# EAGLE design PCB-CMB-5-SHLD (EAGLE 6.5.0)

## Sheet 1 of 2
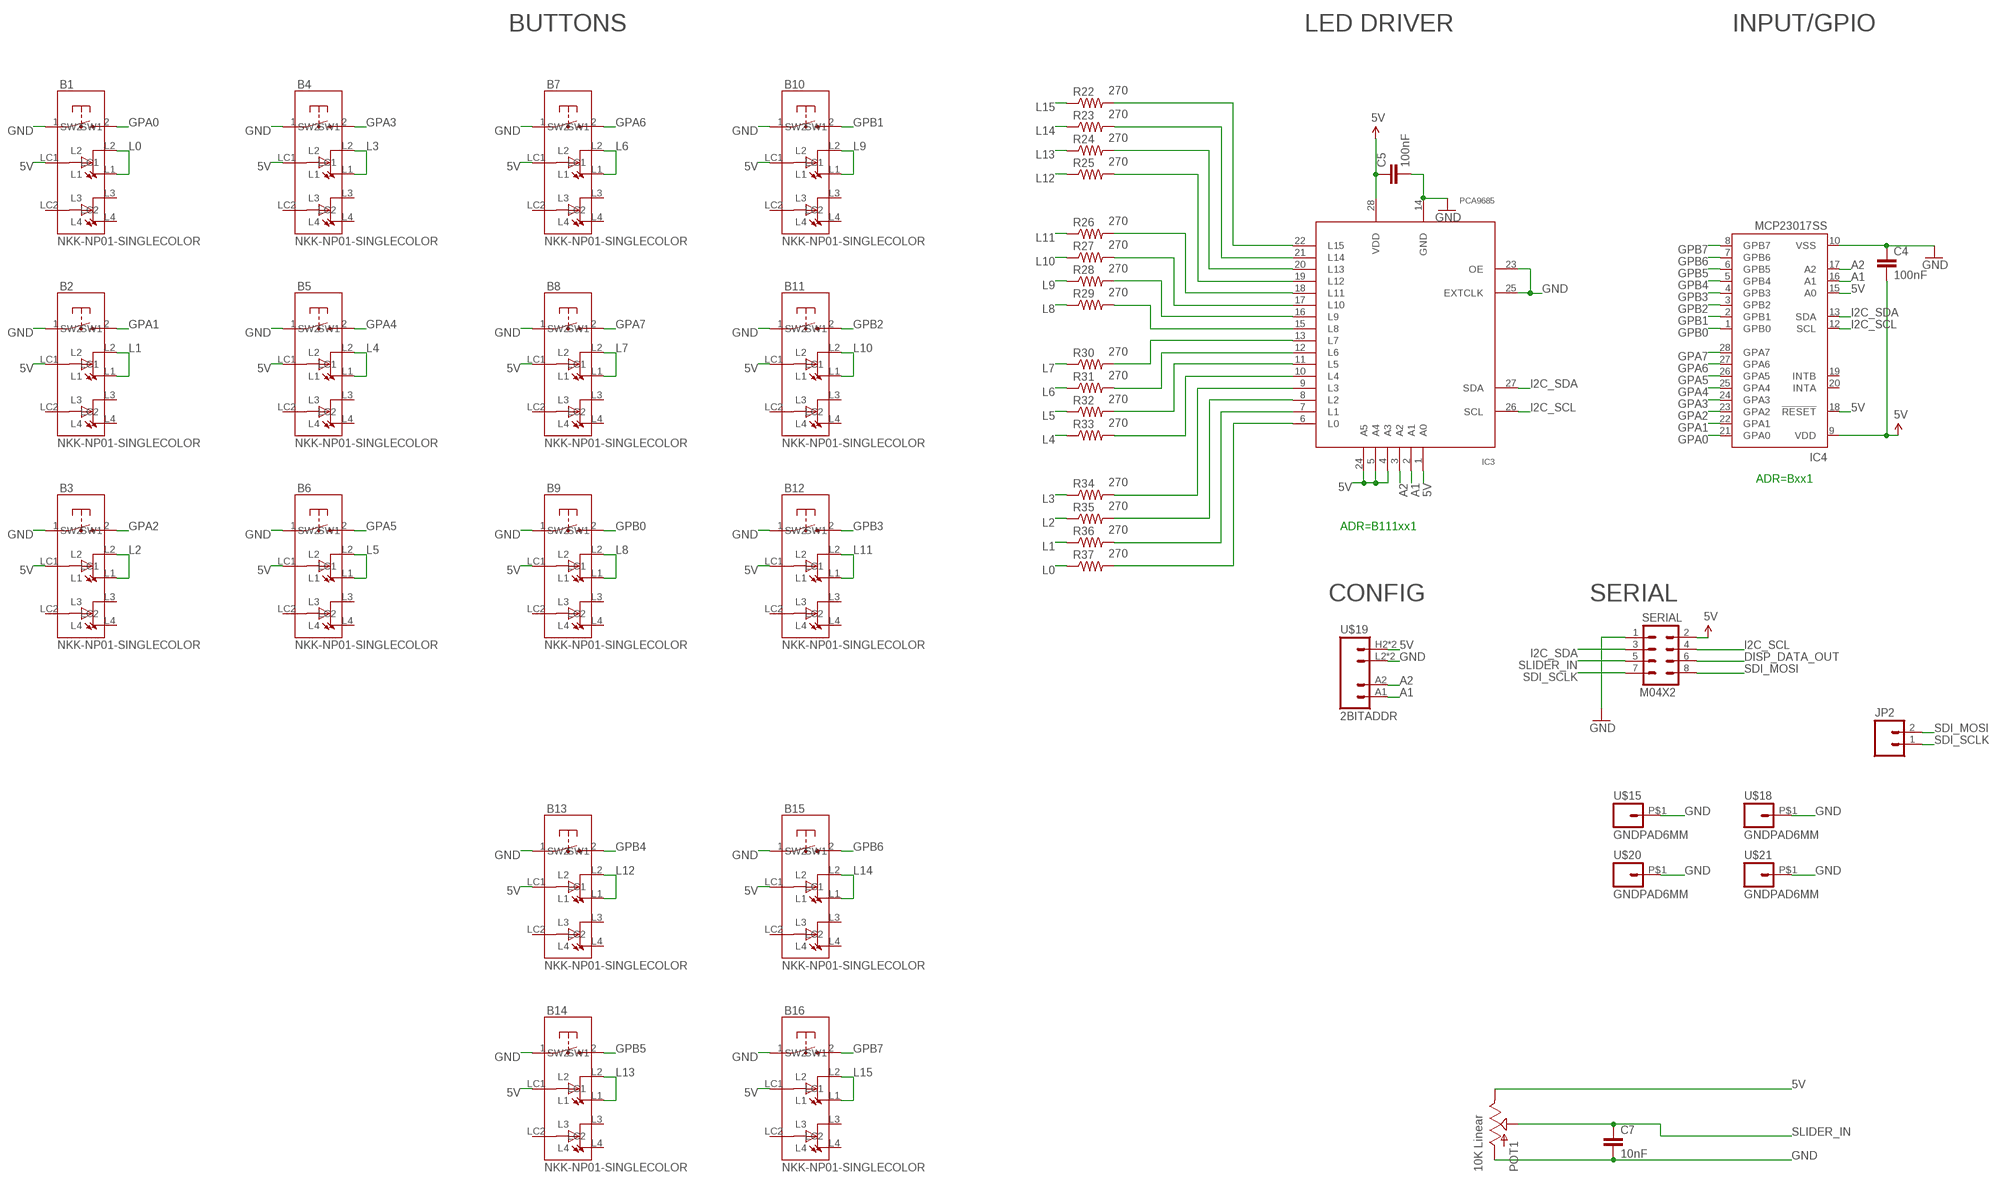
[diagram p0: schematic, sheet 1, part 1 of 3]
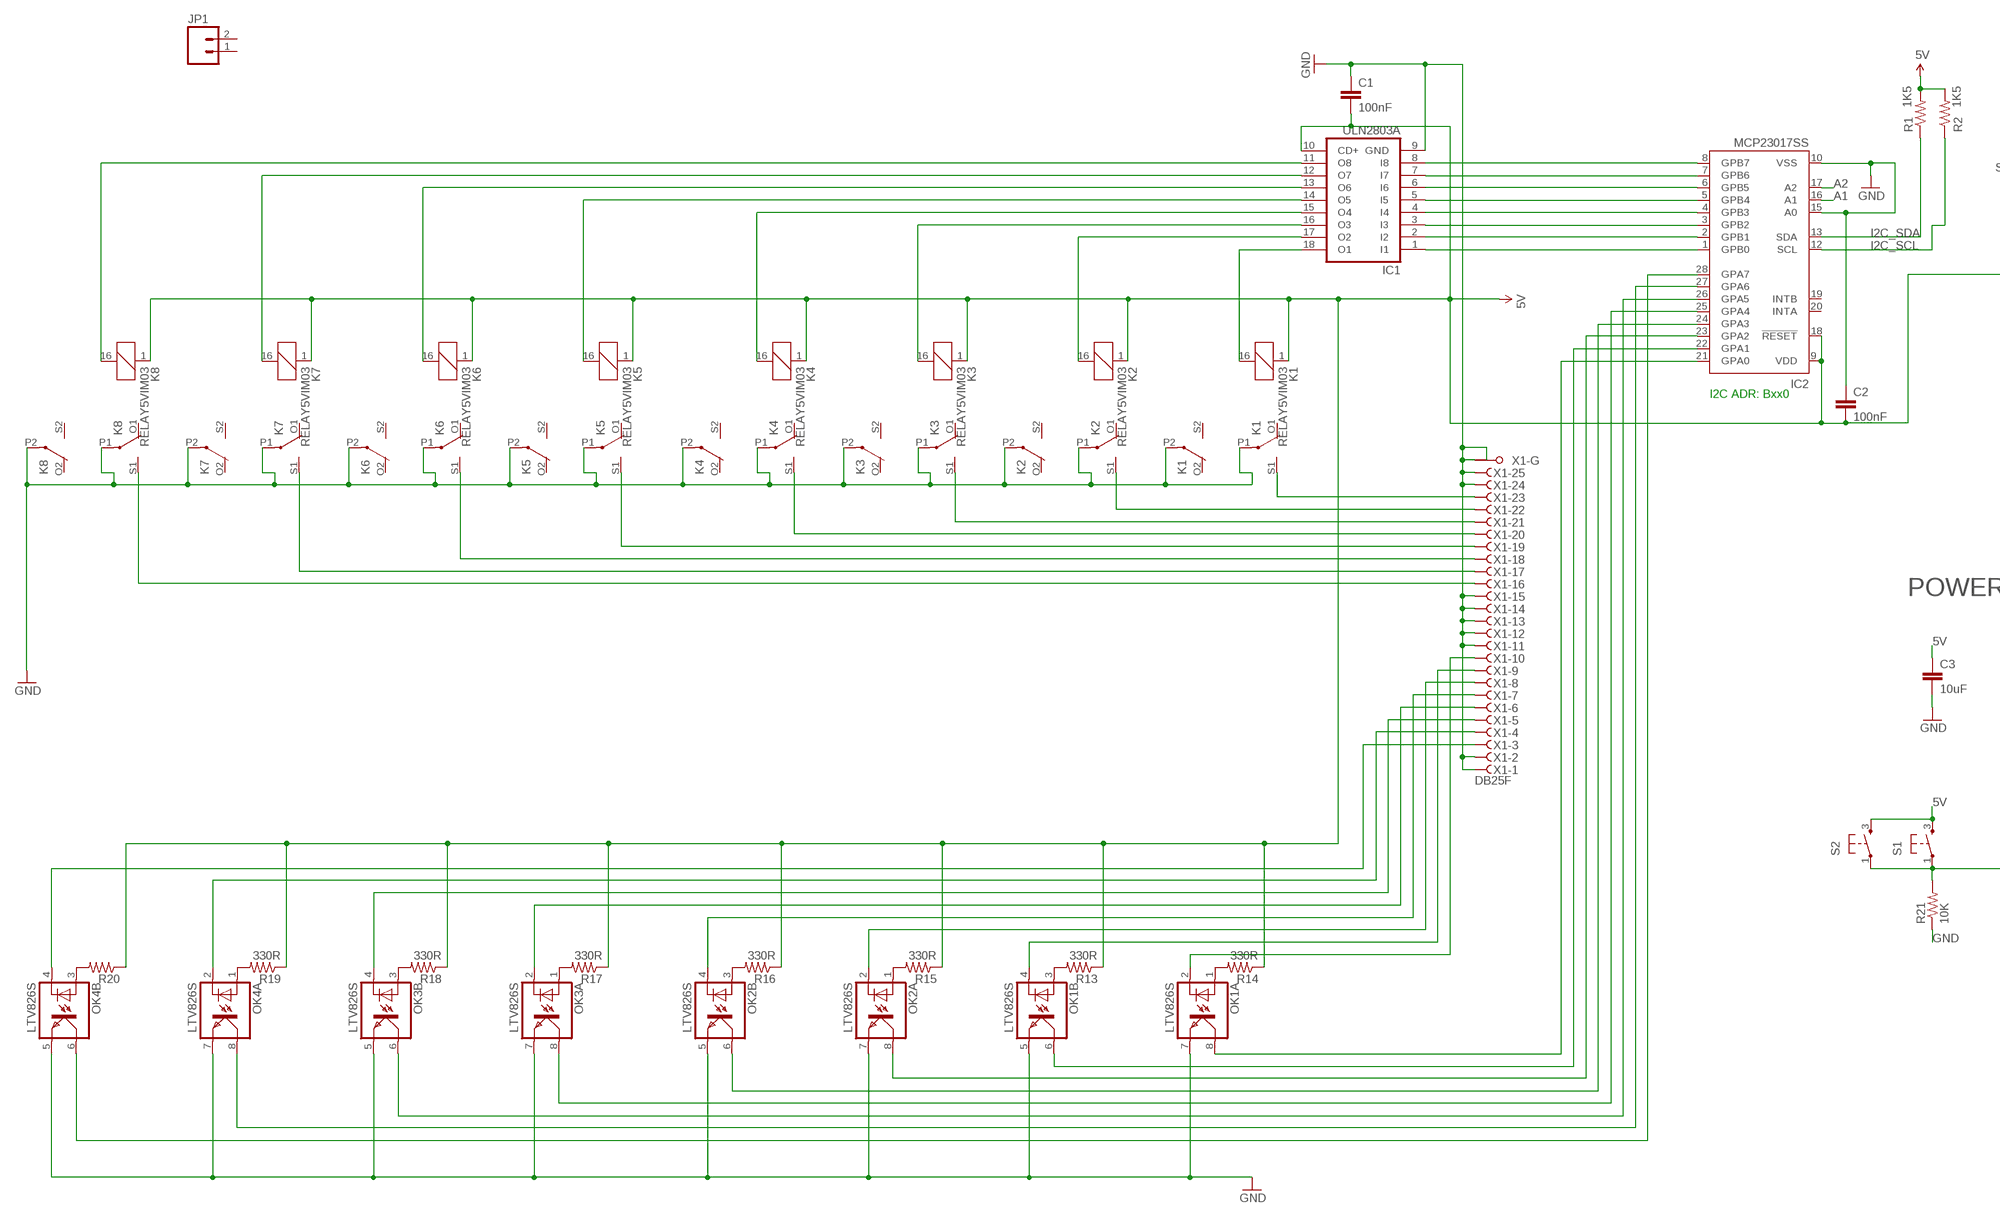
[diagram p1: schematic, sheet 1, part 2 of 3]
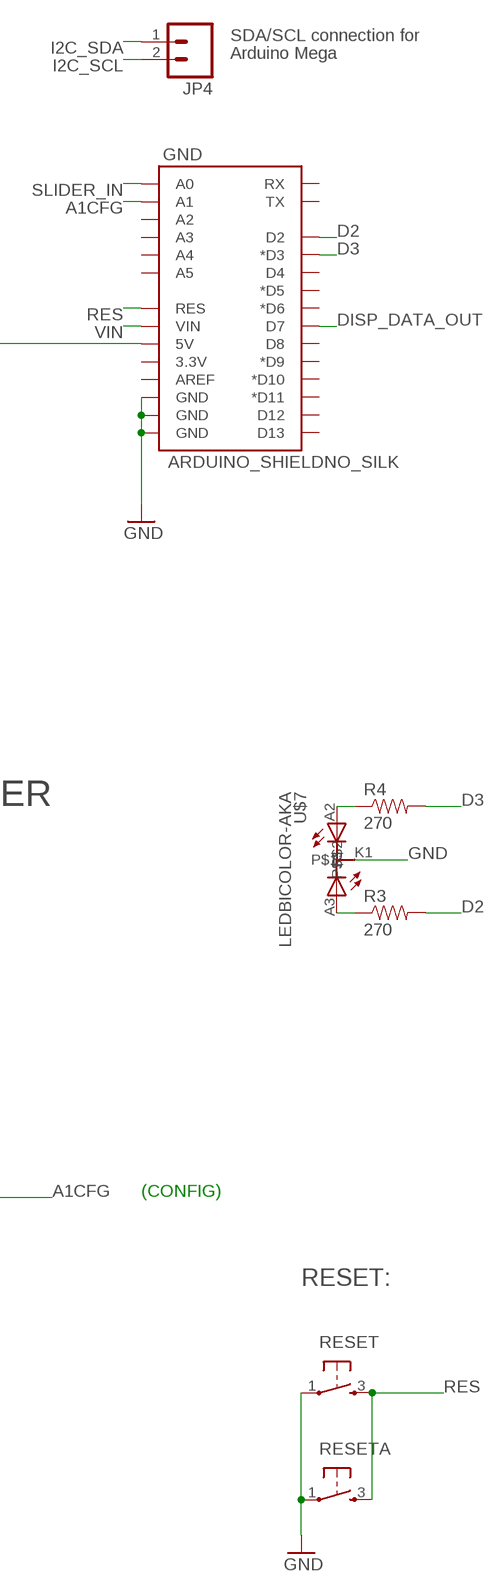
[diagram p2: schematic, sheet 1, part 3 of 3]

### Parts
B1  NKK-NP01-SINGLECOLOR  [NKK-NP01]
B2  NKK-NP01-SINGLECOLOR  [NKK-NP01]
B3  NKK-NP01-SINGLECOLOR  [NKK-NP01]
B4  NKK-NP01-SINGLECOLOR  [NKK-NP01]
B5  NKK-NP01-SINGLECOLOR  [NKK-NP01]
B6  NKK-NP01-SINGLECOLOR  [NKK-NP01]
B7  NKK-NP01-SINGLECOLOR  [NKK-NP01]
B8  NKK-NP01-SINGLECOLOR  [NKK-NP01]
B9  NKK-NP01-SINGLECOLOR  [NKK-NP01]
B10  NKK-NP01-SINGLECOLOR  [NKK-NP01]
B11  NKK-NP01-SINGLECOLOR  [NKK-NP01]
B12  NKK-NP01-SINGLECOLOR  [NKK-NP01]
B13  NKK-NP01-SINGLECOLOR  [NKK-NP01]
B14  NKK-NP01-SINGLECOLOR  [NKK-NP01]
B15  NKK-NP01-SINGLECOLOR  [NKK-NP01]
B16  NKK-NP01-SINGLECOLOR  [NKK-NP01]
C1  100nF  CAP0805  [0805]
C2  100nF  CAP0603-CAP  [0603-CAP]
C3  10uF  CAP0805  [0805]
C4  100nF  CAP0603-CAP  [0603-CAP]
C5  100nF  CAP0603-CAP  [0603-CAP]
C7  10nF  CAP0603-CAP  [0603-CAP]
GND  ARDUINO_SHIELDNO_SILK  [DUEMILANOVE_VIAS]
IC1  ULN2803A  ULN2803ASO18W  [SO18W]
IC2  MCP23017SS  [SSOP28]
IC3  PCA9685  [TSSOP28]
IC4  MCP23017SS  [SSOP28]
JP1  M02PTH  [1X02]
JP2  M02PTH  [1X02]
JP4  M02PTH  [1X02]
K1  RELAY5VIM03  [DS2Y]
K2  RELAY5VIM03  [DS2Y]
K3  RELAY5VIM03  [DS2Y]
K4  RELAY5VIM03  [DS2Y]
K5  RELAY5VIM03  [DS2Y]
K6  RELAY5VIM03  [DS2Y]
K7  RELAY5VIM03  [DS2Y]
K8  RELAY5VIM03  [DS2Y]
OK1  LTV826S  [DIL8-SMD]
OK2  LTV826S  [DIL8-SMD]
OK3  LTV826S  [DIL8-SMD]
OK4  LTV826S  [DIL8-SMD]
POT1  10K Linear  SLIDER20  [SLIDER20]
R1  1K5  RESISTOR0603-RES  [0603-RES]
R2  1K5  RESISTOR0603-RES  [0603-RES]
R3  270  RESISTOR0603-RES  [0603-RES]
R4  270  RESISTOR0603-RES  [0603-RES]
R13  330R  RESISTOR0603-RES  [0603-RES]
R14  330R  RESISTOR0603-RES  [0603-RES]
R15  330R  RESISTOR0603-RES  [0603-RES]
R16  330R  RESISTOR0603-RES  [0603-RES]
R17  330R  RESISTOR0603-RES  [0603-RES]
R18  330R  RESISTOR0603-RES  [0603-RES]
R19  330R  RESISTOR0603-RES  [0603-RES]
R20  RESISTOR0603-RES  [0603-RES]
R21  10K  RESISTOR0603-RES  [0603-RES]
R22  270  RESISTOR0603-RES  [0603-RES]
R23  270  RESISTOR0603-RES  [0603-RES]
R24  270  RESISTOR0603-RES  [0603-RES]
R25  270  RESISTOR0603-RES  [0603-RES]
R26  270  RESISTOR0603-RES  [0603-RES]
R27  270  RESISTOR0603-RES  [0603-RES]
R28  270  RESISTOR0603-RES  [0603-RES]
R29  270  RESISTOR0603-RES  [0603-RES]
R30  270  RESISTOR0603-RES  [0603-RES]
R31  270  RESISTOR0603-RES  [0603-RES]
R32  270  RESISTOR0603-RES  [0603-RES]
R33  270  RESISTOR0603-RES  [0603-RES]
R34  270  RESISTOR0603-RES  [0603-RES]
R35  270  RESISTOR0603-RES  [0603-RES]
R36  270  RESISTOR0603-RES  [0603-RES]
R37  270  RESISTOR0603-RES  [0603-RES]
RESET  TAC_SWITCH  [PUSHBUTTON]
RESETA  TAC_SWITCH  [PUSHBUTTON]
S1  TAC_SWITCH  [PUSHBUTTON]
S2  TAC_SWITCH  [PUSHBUTTON]
SERIAL  M04X2  [2X4]
U$7  LEDBICOLOR-AKA  [LED5MM-BICOLOR]
U$15  GNDPAD6MM  [3.2MMPAD6MM]
U$18  GNDPAD6MM  [3.2MMPAD6MM]
U$19  2BITADDR  [2BITADDR]
U$20  GNDPAD6MM  [3.2MMPAD6MM]
U$21  GNDPAD6MM  [3.2MMPAD6MM]
X1  DB25F  F25HPS  [F25HP]

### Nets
5V [PWR]: B1.LC1 B2.LC1 B3.LC1 B4.LC1 B5.LC1 B6.LC1 B7.LC1 B8.LC1 B9.LC1 B10.LC1 B11.LC1 B12.LC1 B13.LC1 B14.LC1 B15.LC1 B16.LC1 C1.2 C2.2 C3.1 C4.2 C5.1 GND.5V IC1.10(CD+) IC2.9(VDD) IC2.18(!RESET) IC3.1(A0) IC3.4(A3) IC3.5(A4) IC3.24(A5) IC3.28(VDD) IC4.9(VDD) IC4.15(A0) IC4.18(!RESET) K1.1 K2.1 K3.1 K4.1 K5.1 K6.1 K7.1 K8.1 POT1.1(E) R1.2 R2.2 R13.1 R14.1 R15.1 R16.1 R17.1 R18.1 R19.1 R20.1 S1.3 S2.3 SERIAL.2 U$19.H2(VCC) U$19.H3(VCC)
A1: IC2.16(A1) IC3.2(A1) IC4.16(A1) U$19.A1
A1CFG: GND.A1 R21.2 S1.1 S2.1
A2: IC2.17(A2) IC3.3(A2) IC4.17(A2) U$19.A2
D2: GND.D2 R3.2
D3: GND.D3(*D3) R4.2
DISP_DATA_OUT: GND.D7 SERIAL.6
GND [PWR]: B1.1(SW1) B2.1(SW1) B3.1(SW1) B4.1(SW1) B5.1(SW1) B6.1(SW1) B7.1(SW1) B8.1(SW1) B9.1(SW1) B10.1(SW1) B11.1(SW1) B12.1(SW1) B13.1(SW1) B14.1(SW1) B15.1(SW1) B16.1(SW1) C1.1 C2.1 C3.2 C4.1 C5.2 C7.2 GND.GND@0(GND) GND.GND@1(GND) GND.GND@2(GND) IC1.9(GND) IC2.10(VSS) IC2.15(A0) IC3.14(GND) IC3.23(OE) IC3.25(EXTCLK) IC4.10(VSS) K1.P1(2:P) K1.P2(3:P) K2.P1(2:P) K2.P2(3:P) K3.P1(2:P) K3.P2(3:P) K4.P1(2:P) K4.P2(3:P) K5.P1(2:P) K5.P2(3:P) K6.P1(2:P) K6.P2(3:P) K7.P1(2:P) K7.P2(3:P) K8.P1(2:P) K8.P2(3:P) OK1.5(B:EMIT) OK1.7(A:EMIT) OK2.5(B:EMIT) OK2.7(A:EMIT) OK3.5(B:EMIT) OK3.7(A:EMIT) OK4.5(B:EMIT) OK4.7(A:EMIT) POT1.3(A) R21.1 RESET.1 RESETA.1 SERIAL.1 U$7.K1 U$15.P$1 U$18.P$1 U$19.L2(GND) U$19.L3(GND) U$20.P$1 U$21.P$1 X1.1(-1:F) X1.2(-2:F) X1.11(-11:F) X1.12(-12:F) X1.13(-13:F) X1.14(-14:F) X1.15(-15:F) X1.24(-24:F) X1.25(-25:F) X1.G1(-G:G1) X1.G2(-G:G2)
GPA0: B1.2(SW2) IC4.21(GPA0)
GPA1: B2.2(SW2) IC4.22(GPA1)
GPA2: B3.2(SW2) IC4.23(GPA2)
GPA3: B4.2(SW2) IC4.24(GPA3)
GPA4: B5.2(SW2) IC4.25(GPA4)
GPA5: B6.2(SW2) IC4.26(GPA5)
GPA6: B7.2(SW2) IC4.27(GPA6)
GPA7: B8.2(SW2) IC4.28(GPA7)
GPB0 [PWR]: B9.2(SW2) IC4.1(GPB0)
GPB1: B10.2(SW2) IC4.2(GPB1)
GPB2: B11.2(SW2) IC4.3(GPB2)
GPB3: B12.2(SW2) IC4.4(GPB3)
GPB4: B13.2(SW2) IC4.5(GPB4)
GPB5: B14.2(SW2) IC4.6(GPB5)
GPB6: B15.2(SW2) IC4.7(GPB6)
GPB7: B16.2(SW2) IC4.8(GPB7)
I2C_SCL: IC2.12(SCL) IC3.26(SCL) IC4.12(SCL) JP4.2 R2.1 SERIAL.4
I2C_SDA: IC2.13(SDA) IC3.27(SDA) IC4.13(SDA) JP4.1 R1.1 SERIAL.3
L0: B1.L1 B1.L2 R37.1
L1: B2.L1 B2.L2 R36.1
L2: B3.L1 B3.L2 R35.1
L3: B4.L1 B4.L2 R34.1
L4: B5.L1 B5.L2 R33.1
L5: B6.L1 B6.L2 R32.1
L6: B7.L1 B7.L2 R31.1
L7: B8.L1 B8.L2 R30.1
L8: B9.L1 B9.L2 R29.1
L9: B10.L1 B10.L2 R28.1
L10: B11.L1 B11.L2 R27.1
L11: B12.L1 B12.L2 R26.1
L12: B13.L1 B13.L2 R25.1
L13: B14.L1 B14.L2 R24.1
L14: B15.L1 B15.L2 R23.1
L15: B16.L1 B16.L2 R22.1
N$1 [RELAY LINES]: K1.S1(2:S) X1.23(-23:F)
N$2: IC3.13(L7) R30.2
N$4: IC1.18(O1) K1.16
N$5: IC1.1(I1) IC2.1(GPB0)
N$6 [RELAY LINES]: K2.S1(2:S) X1.22(-22:F)
N$7: R4.1 U$7.A2
N$9: IC1.17(O2) K2.16
N$10 [RELAY LINES]: K3.S1(2:S) X1.21(-21:F)
N$11: R3.1 U$7.A3
N$13: IC1.16(O3) K3.16
N$14 [RELAY LINES]: K4.S1(2:S) X1.20(-20:F)
N$17: IC1.15(O4) K4.16
N$18 [RELAY LINES]: K5.S1(2:S) X1.19(-19:F)
N$19: IC3.12(L6) R31.2
N$21: IC1.14(O5) K5.16
N$22 [RELAY LINES]: K6.S1(2:S) X1.18(-18:F)
N$23: IC3.11(L5) R32.2
N$25: IC1.13(O6) K6.16
N$26 [RELAY LINES]: K7.S1(2:S) X1.17(-17:F)
N$29: IC1.12(O7) K7.16
N$30 [RELAY LINES]: K8.S1(2:S) X1.16(-16:F)
N$31: IC3.10(L4) R33.2
N$33: IC1.11(O8) K8.16
N$34: IC1.2(I2) IC2.2(GPB1)
N$35: IC1.3(I3) IC2.3(GPB2)
N$36: IC1.4(I4) IC2.4(GPB3)
N$37: IC1.5(I5) IC2.5(GPB4)
N$38: IC1.6(I6) IC2.6(GPB5)
N$39: IC1.7(I7) IC2.7(GPB6)
N$40: IC1.8(I8) IC2.8(GPB7)
N$47: OK1.3(B:A) R13.2
N$48: OK1.1(A:A) R14.2
N$49 [INput lines]: OK1.2(A:C) X1.10(-10:F)
N$50: OK2.1(A:A) R15.2
N$51: IC2.21(GPA0) OK1.8(A:COL)
N$52: OK2.3(B:A) R16.2
N$53: OK3.1(A:A) R17.2
N$54: OK3.3(B:A) R18.2
N$55 [INput lines]: OK3.2(A:C) X1.6(-6:F)
N$56: OK4.1(A:A) R19.2
N$57: OK4.3(B:A) R20.2
N$58: IC3.9(L3) R34.2
N$59: IC3.8(L2) R35.2
N$60 [INput lines]: OK1.4(B:C) X1.9(-9:F)
N$61 [INput lines]: OK2.2(A:C) X1.8(-8:F)
N$62 [INput lines]: OK2.4(B:C) X1.7(-7:F)
N$63: IC2.28(GPA7) OK4.6(B:COL)
N$64 [INput lines]: OK3.4(B:C) X1.5(-5:F)
N$65 [INput lines]: OK4.2(A:C) X1.4(-4:F)
N$66 [INput lines]: OK4.4(B:C) X1.3(-3:F)
N$67: IC3.7(L1) R36.2
N$68: IC2.22(GPA1) OK1.6(B:COL)
N$69: IC2.23(GPA2) OK2.8(A:COL)
N$70: IC2.24(GPA3) OK2.6(B:COL)
N$71: IC2.25(GPA4) OK3.8(A:COL)
N$72: IC2.26(GPA5) OK3.6(B:COL)
N$73: IC2.27(GPA6) OK4.8(A:COL)
N$74: IC3.6(L0) R37.2
N$75: IC3.15(L8) R29.2
N$76: IC3.16(L9) R28.2
N$77: IC3.17(L10) R27.2
N$78: IC3.18(L11) R26.2
N$79: IC3.19(L12) R25.2
N$80: IC3.20(L13) R24.2
N$81: IC3.21(L14) R23.2
N$82: IC3.22(L15) R22.2
RES: GND.RES RESET.3 RESETA.3
SDI_MOSI: JP2.2 SERIAL.8
SDI_SCLK: JP2.1 SERIAL.7
SLIDER_IN: C7.1 GND.A0 POT1.2A(S) SERIAL.5
VIN: GND.VIN
Unconnected: B1.L3 B1.L4 B1.LC2 B2.L3 B2.L4 B2.LC2 B3.L3 B3.L4 B3.LC2 B4.L3 B4.L4 B4.LC2 B5.L3 B5.L4 B5.LC2 B6.L3 B6.L4 B6.LC2 B7.L3 B7.L4 B7.LC2 B8.L3 B8.L4 B8.LC2 B9.L3 B9.L4 B9.LC2 B10.L3 B10.L4 B10.LC2 B11.L3 B11.L4 B11.LC2 B12.L3 B12.L4 B12.LC2 B13.L3 B13.L4 B13.LC2 B14.L3 B14.L4 B14.LC2 B15.L3 B15.L4 B15.LC2 B16.L3 B16.L4 B16.LC2 GND.3.3V GND.A2 GND.A3 GND.A4 GND.A5 GND.AREF GND.D4 GND.D5(*D5) GND.D6(*D6) GND.D8 GND.D9(*D9) GND.D10(*D10) GND.D11(*D11) GND.D12 GND.D13 GND.RX GND.TX IC2.19(INTB) IC2.20(INTA) IC4.19(INTB) IC4.20(INTA) JP1.1 JP1.2 K1.O1(2:O) K1.O2(3:O) K1.S2(3:S) K2.O1(2:O) K2.O2(3:O) K2.S2(3:S) K3.O1(2:O) K3.O2(3:O) K3.S2(3:S) K4.O1(2:O) K4.O2(3:O) K4.S2(3:S) K5.O1(2:O) K5.O2(3:O) K5.S2(3:S) K6.O1(2:O) K6.O2(3:O) K6.S2(3:S) K7.O1(2:O) K7.O2(3:O) K7.S2(3:S) K8.O1(2:O) K8.O2(3:O) K8.S2(3:S)

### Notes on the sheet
- BUTTONS | LED DRIVER | INPUT/GPIO
- ADR=Bxx1
- ADR=B111xx1
- CONFIG | SERIAL
- SDA/SCL connection for
- Arduino Mega
- I2C ADR: Bxx0
- POWER
- (CONFIG)
- RESET:

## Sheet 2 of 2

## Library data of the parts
B1-B16 = SKAARHOJ:NKK-NP01-SINGLECOLOR
C1-C5 C7 = SparkFun:CAP: Capacitor
GND = SparkFun:ARDUINO_SHIELD
IC1 = uln-udn:ULN2803A: DRIVER ARRAY
IC2 IC4 = microchip:MCP23017: http://ww1.microchip.com/downloads/en/DeviceDoc/21952a.pdf Source: http://ww1.microchip.com/downloads/en/DeviceDoc/21952a.pdf; MF: MICROCHIP; MPN: MCP23017-E/SS; OC_FARNELL: 1467674; OC_NEWARK: 31K2960
IC3 = wsmith:PCA9685
JP1 JP2 JP4 = SparkFun:M02: Header 2
K1-K8 = SKAARHOJ:RELAY5V: RELAY 2 x switch, AxiCom 150 mW 5V
OK1-OK4 = optocoupler:LTV826: OPTO COUPLER Source: LITEON, LTV816.pdf; OC_FARNELL: unknown; OC_NEWARK: unknown
POT1 = SKAARHOJ:SLIDER
R1-R4 R13-R37 = SparkFun:RESISTOR: Resistor
RESET RESETA S1 S2 = SKAARHOJ:TAC_SWITCH: Momentary Switch
SERIAL = SparkFun:M04X2
U$7 = SKAARHOJ:LEDBICOLOR-AKA
U$15 U$18 U$20 U$21 = SKAARHOJ:GNDPAD
U$19 = SKAARHOJ:2BITADDR
X1 = con-subd:F25HPS: SUB-D; OC_FARNELL: unknown; OC_NEWARK: unknown

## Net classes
0 default: width 0.203 mm, drill 0.406 mm, clearance 0.203 mm
1 PWR: width 0.406 mm, drill 0.61 mm, clearance 0.203 mm
2 RELAY LINES: width 0.305 mm, clearance 0.203 mm
3 INput lines: clearance 0.203 mm

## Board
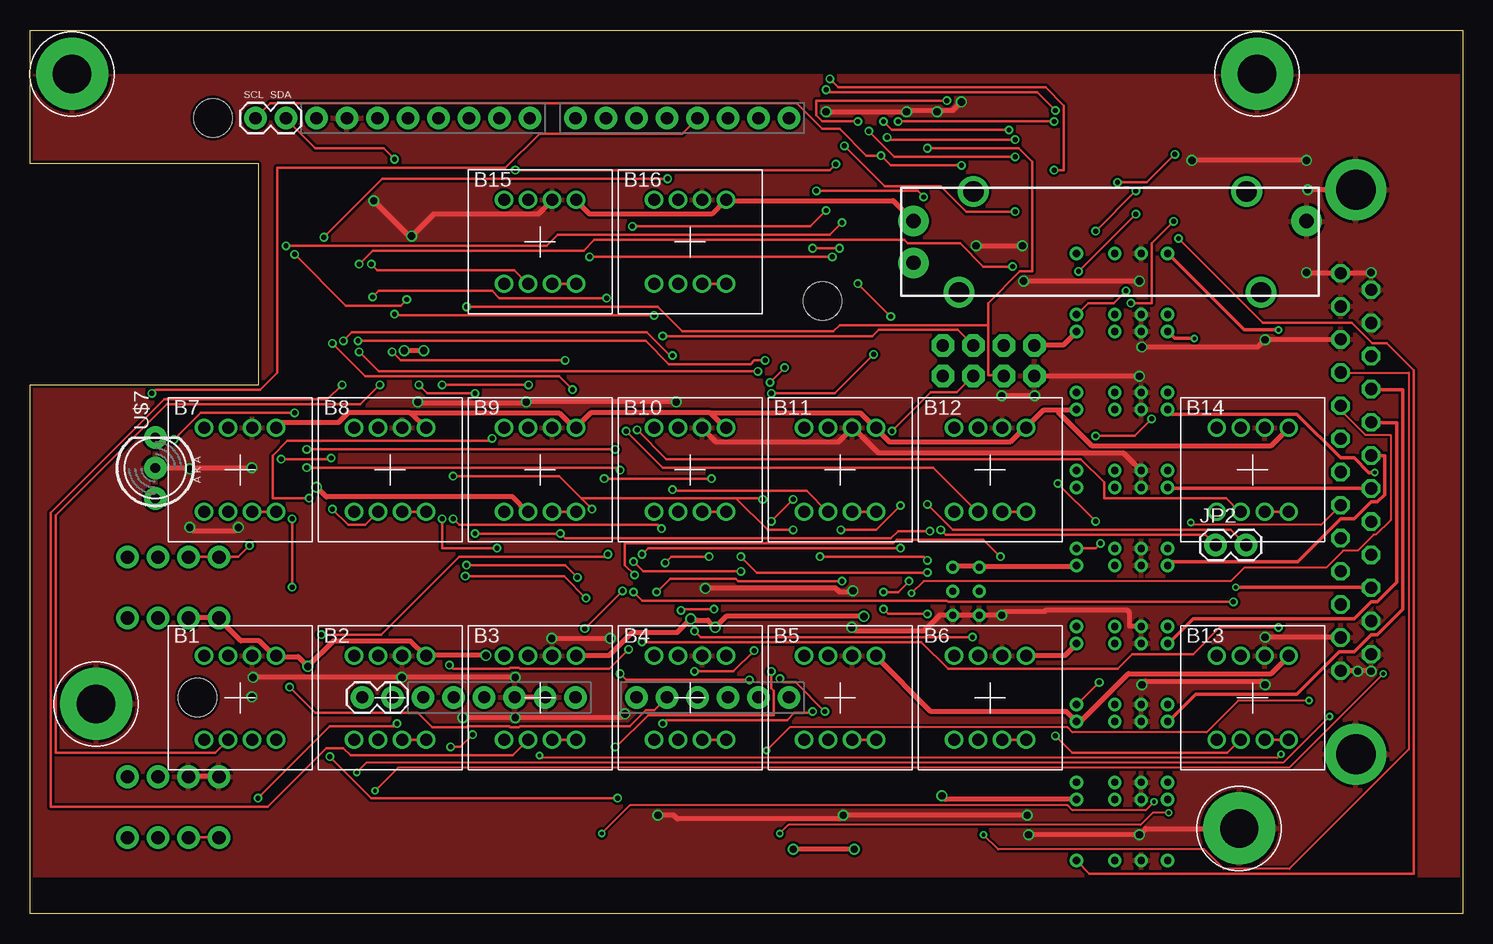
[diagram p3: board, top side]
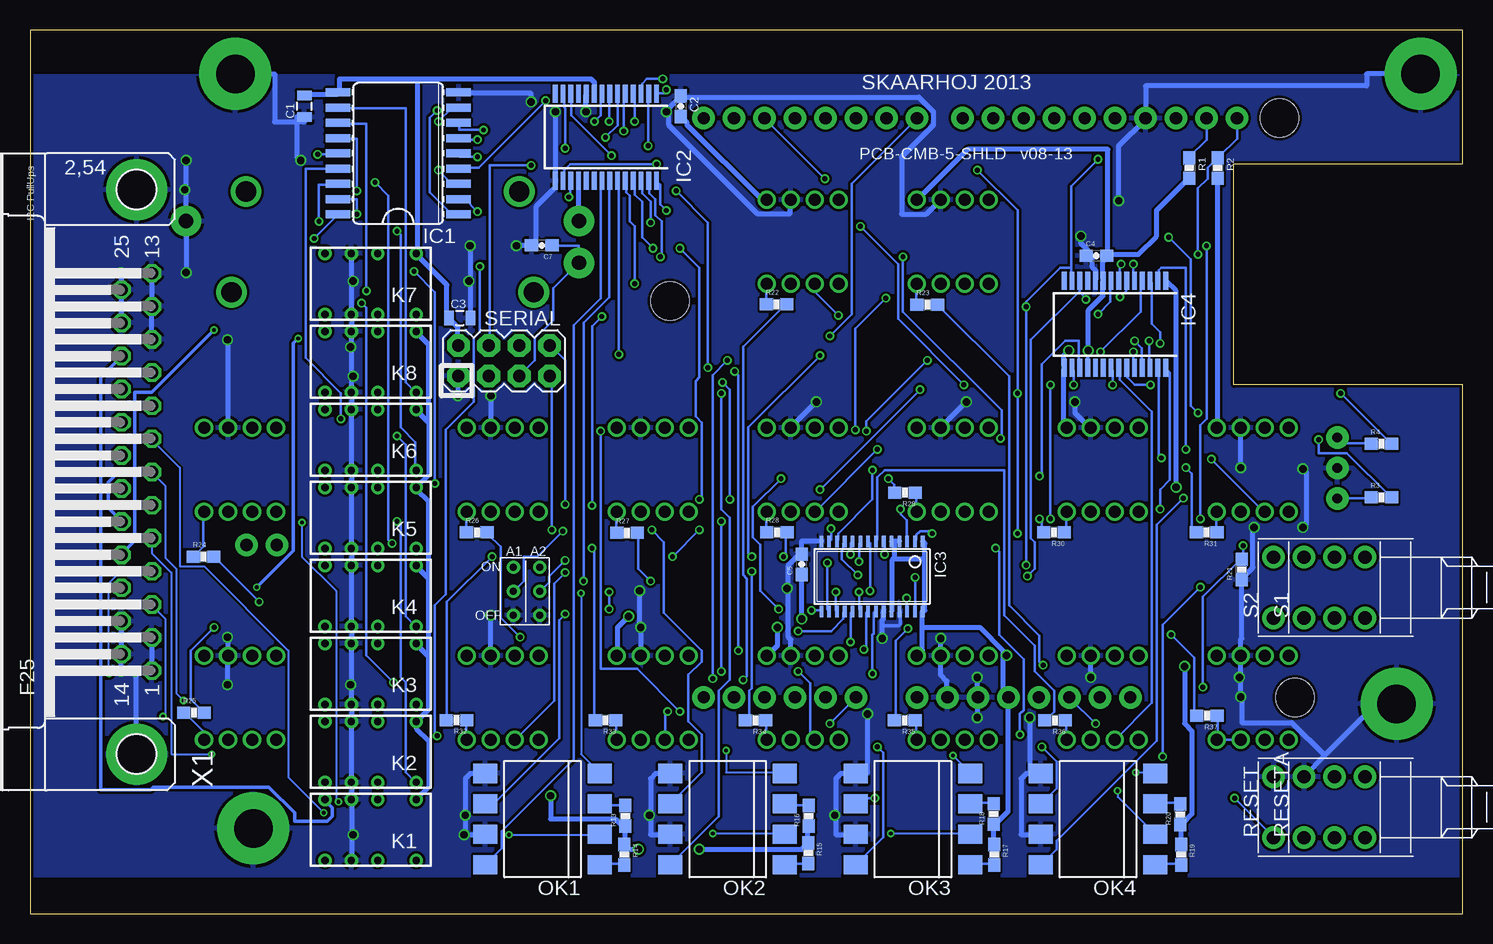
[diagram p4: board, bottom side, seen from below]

Size 119.38 x 73.66 mm. Coordinates in mm from the lower left corner, seen from the top.
Outline: 0,0 0,44.09 19.05,44.09 19.05,62.5 0,62.5 0,73.66 119.38,73.66 119.38,0 0,0
Copper layers (1*16): Top 0.035mm / dielectric 1.5mm / Bottom 0.035mm
Design rules "Fusion_eagle_rule_v1.1": minimum track width 6mil, minimum drill 12mil, track to track 6mil, track to pad 6mil, pad to pad 6mil, via to via 6mil, smd to smd 0mil, copper to edge 10mil, drill to drill 10mil, minimum pad ring 10mil, minimum via ring 6mil, stop-mask expansion 2mil, vias tented up to drill 100mil, thermal gap 10mil
Holes 3.2 mm at 66.04,51.07 15.24,66.31 13.97,18.05
tRestrict: area 0,0 to 120,3; area 0,70 to 120,74
bRestrict: area 0,70 to 120,74; area 0,0 to 120,3

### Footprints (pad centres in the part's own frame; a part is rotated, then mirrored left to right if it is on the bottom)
NKK-NP01 = drill 1: 1 1,3.5; 2 -1,-3.5; L1 3,-3.5; L2 1,-3.5; L3 -1,3.5; L4 -3,3.5; LC1 3,3.5; LC2 -3,-3.5
0805 = smd 0.8 x 1.2: 1 -0.9,0; 2 0.9,0
0603-CAP = smd 1.1 x 1: 1 -0.85,0; 2 0.85,0
DUEMILANOVE_VIAS = drill 1.016 pad 1.88: 3.3V 50.8,13.97; 5V 50.8,16.51; A0 50.8,29.21; A1 50.8,31.75; A2 50.8,34.29; A3 50.8,36.83; A4 50.8,39.37; A5 50.8,41.91; AREF 2.54,2.54; D2 2.54,36.83; D3 2.54,34.29; D4 2.54,31.75; D5 2.54,29.21; D6 2.54,26.67; D7 2.54,24.13; D8 2.54,20.32; D9 2.54,17.78; D10 2.54,15.24; D11 2.54,12.7; D12 2.54,10.16; D13 2.54,7.62; GND@0 50.8,19.05; GND@1 50.8,21.59; GND@2 2.54,5.08; RES 50.8,11.43; RX 2.54,41.91; TX 2.54,39.37; VIN 50.8,24.13
SO18W = smd 0.66 x 2.032: 1 -5.08,-5.029; 2 -3.81,-5.029; 3 -2.54,-5.029; 4 -1.27,-5.029; 5 0,-5.029; 6 1.27,-5.029; 7 2.54,-5.029; 8 3.81,-5.029; 9 5.08,-5.029; 10 5.08,5.029; 11 3.81,5.029; 12 2.54,5.029; 13 1.27,5.029; 14 0,5.029; 15 -1.27,5.029; 16 -2.54,5.029; 17 -3.81,5.029; 18 -5.08,5.029
SSOP28 = smd 0.4 x 1.5: 1 -4.225,-3.625; 2 -3.575,-3.625; 3 -2.925,-3.625; 4 -2.275,-3.625; 5 -1.625,-3.625; 6 -0.975,-3.625; 7 -0.325,-3.625; 8 0.325,-3.625; 9 0.975,-3.625; 10 1.625,-3.625; 11 2.275,-3.625; 12 2.925,-3.625; 13 3.575,-3.625; 14 4.225,-3.625; 15 4.225,3.625; 16 3.575,3.625; 17 2.925,3.625; 18 2.275,3.625; 19 1.625,3.625; 20 0.975,3.625; 21 0.325,3.625; 22 -0.325,3.625; 23 -0.975,3.625; 24 -1.625,3.625; 25 -2.275,3.625; 26 -2.925,3.625; 27 -3.575,3.625; 28 -4.225,3.625
TSSOP28 = smd 0.305 x 0.991: 1 -4.225,-2.918; 2 -3.575,-2.918; 3 -2.925,-2.918; 4 -2.275,-2.918; 5 -1.625,-2.918; 6 -0.975,-2.918; 7 -0.325,-2.918; 8 0.325,-2.918; 9 0.975,-2.918; 10 1.625,-2.918; 11 2.275,-2.918; 12 2.925,-2.918; 13 3.575,-2.918; 14 4.225,-2.918; 15 4.225,2.918; 16 3.575,2.918; 17 2.925,2.918; 18 2.275,2.918; 19 1.625,2.918; 20 0.975,2.918; 21 0.325,2.918; 22 -0.325,2.918; 23 -0.975,2.918; 24 -1.625,2.918; 25 -2.275,2.918; 26 -2.925,2.918; 27 -3.575,2.918; 28 -4.225,2.918
1X02 = drill 1.016 pad 1.88: 1 0,0; 2 2.54,0
DS2Y = drill 0.6: 1 1.2,0.46; 16 1.2,5.54; O1 4.4,0.46; O2 4.4,5.54; P1 6.6,0.46; P2 6.6,5.54; S1 8.8,0.46; S2 8.8,5.54
DIL8-SMD = smd 1.6 x 2: 1 -3.81,-4.77; 2 -1.27,-4.77; 3 1.27,-4.77; 4 3.81,-4.77; 5 3.81,4.77; 6 1.27,4.77; 7 -1.27,4.77; 8 -3.81,4.77
SLIDER20 = drill 1.194 pad 2.54: 1 -16.383,1.74; 2A -16.383,-1.74; 3 16.383,1.74 | drill 1.702: P$1 -11.392,4.191; P$2 11.392,4.191; P$3 12.598,-4.191; P$4 -12.598,-4.191
0603-RES = smd 1.1 x 1: 1 -0.85,0; 2 0.85,0
PUSHBUTTON = drill 1.1 pad 1.88: 1 2.54,2.54; 2 2.54,-2.54; 3 -2.54,2.54; 4 -2.54,-2.54
2X4 = drill 1.016 pad 1.88 octagon: 1 -3.81,-1.27; 2 -3.81,1.27; 3 -1.27,-1.27; 4 -1.27,1.27; 5 1.27,-1.27; 6 1.27,1.27; 7 3.81,-1.27; 8 3.81,1.27
LED5MM-BICOLOR = drill 0.813 pad 1.88: A2 2.54,0; A3 -2.54,0; K1 0,0
3.2MMPAD6MM = drill 3.2 pad 6: P$1 0,0
2BITADDR = drill 0.6: A1 0,0; A2 2.2,0; H2 0,2; H3 2.2,2; L2 0,-2; L3 2.2,-2
F25HP = drill 1.016 octagon: 1 -16.561,-1.27; 2 -13.792,-1.27; 3 -11.049,-1.27; 4 -8.28,-1.27; 5 -5.512,-1.27; 6 -2.769,-1.27; 7 0,-1.27; 8 2.769,-1.27; 9 5.512,-1.27; 10 8.28,-1.27; 11 11.049,-1.27; 12 13.792,-1.27; 13 16.561,-1.27; 14 -15.189,1.27; 15 -12.421,1.27; 16 -9.652,1.27; 17 -6.909,1.27; 18 -4.14,1.27; 19 -1.372,1.27; 20 1.372,1.27; 21 4.14,1.27; 22 6.909,1.27; 23 9.652,1.27; 24 12.421,1.27; 25 15.189,1.27 | drill 3.302 pad 5.08: G1 -23.52,0; G2 23.52,0

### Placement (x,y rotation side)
B1  17.5,18 0 top
B2  30,18 0 top
B3  42.5,18 0 top
B4  55,18 0 top
B5  67.5,18 0 top
B6  80,18 0 top
B7  17.5,37 0 top
B8  30,37 0 top
B9  42.5,37 0 top
B10  55,37 0 top
B11  67.5,37 0 top
B12  80,37 0 top
B13  101.88,18 0 top
B14  101.88,37 0 top
B15  42.5,56 0 top
B16  55,56 0 top
C1  96.52,67.31 90 bottom
C2  65.15,67.31 270 bottom
C3  83.57,49.66 0 bottom
C4  30.51,54.86 0 bottom
C5  55.07,29.13 90 bottom
C7  76.73,55.71 180 bottom
GND  21.34,68.85 270 top
IC1  88.7,63.38 90 bottom
IC2  71.39,64.73 180 bottom
IC3  49.21,28.12 180 bottom
IC4  28.97,49.12 180 bottom
JP1  27.69,18.05 0 top
JP2  98.81,30.75 0 top
JP4  21.34,66.31 180 top
K1  86,10 180 bottom
K2  86,16.5 180 bottom
K3  86,23 180 bottom
K4  86,29.5 180 bottom
K5  86,36 180 bottom
K6  86,42.5 180 bottom
K7  86,55.5 180 bottom
K8  86,49 180 bottom
OK1  76.67,7.9 90 bottom
OK2  61.24,7.9 90 bottom
OK3  45.81,7.9 90 bottom
OK4  30.38,7.9 90 bottom
POT1  90,56 0 top
R1  22.77,62.15 270 bottom
R2  20.4,62.15 270 bottom
R3  6.76,34.71 0 bottom
R4  6.76,39.17 0 bottom
R13  69.76,8.18 90 bottom
R14  69.86,4.93 270 bottom
R15  54.53,5.06 270 bottom
R16  54.47,8.18 90 bottom
R17  39.03,4.93 270 bottom
R18  39.06,8.32 90 bottom
R19  23.46,4.93 270 bottom
R20  23.52,8.3 90 bottom
R21  18.41,28.72 90 bottom
R22  57.16,50.8 0 bottom
R23  44.61,50.77 0 bottom
R24  104.91,29.77 0 bottom
R25  105.72,16.77 0 bottom
R26  82.15,31.79 0 bottom
R27  69.62,31.75 0 bottom
R28  57.14,31.82 0 bottom
R29  46.47,35.11 180 bottom
R30  34.04,31.8 180 bottom
R31  21.32,31.8 180 bottom
R32  83.84,16.16 180 bottom
R33  71.41,16.14 180 bottom
R34  58.93,16.12 180 bottom
R35  46.48,16.12 180 bottom
R36  33.96,16.12 180 bottom
R37  21.31,16.5 180 bottom
RESET  13.21,8.89 90 bottom
RESETA  10.67,8.89 90 bottom
S1  10.67,27.19 90 bottom
S2  13.21,27.19 90 bottom
SERIAL  79.88,46.1 0 bottom
U$7  10.44,37.16 90 top
U$15  100.77,7.12 0 top
U$18  102.26,70 0 top
U$19  79.1,26.89 0 bottom
U$20  5.5,17.5 0 top
U$21  3.5,70 0 top
X1  110.49,36.83 90 bottom

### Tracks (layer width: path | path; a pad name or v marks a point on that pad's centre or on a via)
5V  (via drill 0.61)
  Top 0.406: B15.LC1 45.52,59.44 46.63,58.32 56.79,58.32 57.91,59.44 B16.LC1 58.12,59.44 71.93,59.44 73.56,57.81 POT1.1 | 56.79,41.66 57.91,40.54 B10.LC1 | 56.79,41.66 56.69,41.76 46.74,41.76 45.52,40.54 B9.LC1 45.31,40.54 44.09,41.76 31.9,41.76 31.8,41.66 | 56.79,41.66 56.9,41.76 69.19,41.76 70.41,40.54 B11.LC1 70.61,40.34 71.63,39.32 81.69,39.32 82.8,40.44 B12.LC1 83.01,40.54 84.43,41.96 85.65,41.96 | v32.82,46.94 v31.19,46.94 | 31.8,41.66 32.92,40.54 B8.LC1 | 31.8,41.66 31.7,41.76 26.52,41.76 25.7,40.95 20.93,40.95 20.52,40.54 B7.LC1 | S1.3 13.21,24.69 15.75,24.69 S2.3 15.85,24.49 17.58,22.76 19.1,22.76 20.32,21.54 B1.LC1 20.52,21.44 22.35,21.44 v23.16,20.62 25.3,22.76 31.7,22.76 32.92,21.54 B2.LC1 33.12,21.54 v38,21.54 | B3.LC1 45.52,21.54 48.26,21.54 50.19,23.47 53.95,23.47 v55.07,24.59 55.17,24.49 56.49,24.49 v57.1,23.88 58.01,24.79 v69.49,24.79 | K8.1 87.17,48.46 86.16,47.45 83.72,47.45 SERIAL.2 | 85.65,41.96 87.17,41.96 K6.1 | B14.LC1 104.85,40.44 103.43,39.01 88.49,39.01 85.65,41.86 85.65,41.96 | v68.68,5.38 v63.6,5.38 | U$19.H3 76.91,28.96 79.05,28.96 U$19.H2 79.25,28.96 87.17,28.96 K4.1 | K3.1 87.17,22.45 86.26,21.54 83.01,21.54 B6.LC1 | B5.LC1 70.51,21.44 75.08,16.87 86.36,16.87 87.17,16.05 K2.1 87.38,16.05 87.58,16.05 91.54,20.02 103.43,20.02 104.85,21.44 B13.LC1 | v76,9.86 76.3,9.55 87.17,9.55 K1.1
  Bottom 0.305: v31.19,46.94 31.25,46.94 IC4.18
  Bottom 0.406: IC2.18 73.66,61.06 73.66,57.81 POT1.1 | C2.2 65.13,66.45 64.62,65.94 64.62,65.73 58.42,59.54 58.01,59.54 B16.LC1 | R2.2 20.42,61.27 20.42,40.54 B7.LC1 | R1.2 22.86,61.27 25.5,58.62 25.5,56.49 27.03,54.97 29.57,54.97 29.57,54.86 C4.2 | B8.LC1 33.02,40.54 33.22,40.74 33.22,45.41 IC4.15 33.22,45.62 33.22,46.53 v32.82,46.94 | v31.19,46.94 31.19,50.29 29.97,51.51 29.97,52.73 IC4.9 29.97,52.93 29.97,54.36 29.67,54.66 C4.2 | B15.LC1 45.41,59.54 41.25,63.7 29.57,63.7 29.57,55.07 C4.2 | R19.1 23.47,5.79 23.47,7.42 R20.1 23.37,7.52 22.55,8.33 22.55,15.24 23.16,15.85 v23.16,20.62 | R17.1 39.12,5.79 39.12,7.42 R18.1 38.91,7.52 37.9,8.53 37.9,17.98 GND.5V 37.9,18.19 38.3,18.59 38.3,21.54 | 47.35,31.09 47.55,31.09 IC3.5 | 47.35,31.09 46.94,31.09 IC3.4 | 47.35,29.67 47.55,29.46 47.55,25.3 IC3.24 | 47.35,31.09 47.35,29.67 | 45.01,23.88 45.01,21.95 45.41,21.54 B3.LC1 | 45.01,23.88 45.01,25.2 IC3.28 44.81,25.3 44.81,29.57 | 44.81,29.57 44.81,30.89 44.91,30.99 IC3.1 | v55.07,24.59 55.07,28.25 C5.1 | v57.1,23.88 57.1,22.35 57.91,21.54 B4.LC1 | 44.81,29.57 47.24,29.57 47.35,29.67 | 38.3,21.54 38.3,21.95 40.23,23.88 45.01,23.88 | 38.3,21.54 v38,21.54 | C1.2 96.52,68.28 93.78,68.28 93.78,68.38 IC1.10 93.57,68.58 93.57,69.6 87.07,69.6 | 87.07,69.6 72.64,69.6 72.34,69.29 72.34,68.38 IC2.9 | SERIAL.2 83.72,47.45 83.72,48.87 84.43,49.58 C3.1 84.63,49.78 84.63,52.43 87.17,54.97 K7.1 87.07,55.17 87.07,69.6 | 86.26,41.05 87.17,41.96 K6.1 | 86.26,41.05 86.16,40.95 86.16,36.58 87.17,35.56 K5.1 87.17,35.36 86.16,34.34 86.16,28.14 86.26,28.04 | K8.1 87.17,48.46 86.16,47.45 86.16,41.15 86.26,41.05
  Bottom 0.406: R16.1 54.56,7.32 54.56,5.99 R15.1 54.66,5.79 55.07,5.38 v63.6,5.38 | v68.68,5.38 69.6,5.38 69.6,5.79 R14.1 69.8,5.79 69.8,7.32 R13.1 70,7.32 70.61,7.92 76,7.92 v76,9.86 | K1.1 87.17,9.55 86.16,10.57 86.16,14.43 87.17,15.44 87.17,15.95 K2.1 87.07,16.15 86.16,17.07 86.16,21.44 86.26,21.54 | 86.26,21.54 87.17,22.45 K3.1 | 86.26,28.04 86.16,27.94 86.16,21.64 86.26,21.54 | 86.26,28.04 87.17,28.96 K4.1 | v69.49,24.79 70.41,23.88 70.41,21.54 B5.LC1
A1  (via drill 0.41)
  Top 0.203: v74.98,31.9 72.34,31.9 71.73,31.29 44.6,31.29 v44.2,31.7 v37.08,31.7 | v32.41,44.09 33.12,43.38 v37.08,43.38 | v67.16,62.48 66.65,61.98 v40.44,61.98
  Bottom 0.203: v44.2,31.7 44.2,31.9 45.21,31.9 45.52,31.6 45.52,31.19 45.62,31.09 IC3.2 | v74.98,31.9 77.11,29.77 78.23,29.77 78.23,27.74 79.05,26.92 U$19.A1 | v32.41,44.09 32.41,45.31 32.51,45.41 IC4.16 | v37.08,31.7 v37.08,43.38 37.08,58.62 v40.44,61.98 | v67.16,62.48 74.37,62.48 74.88,61.98 74.88,61.16 IC2.16
A1CFG  (via drill 0.41)
  Top 0.203: v18.29,30.68 17.37,29.77 15.75,29.77 | v21.64,18.9 23.77,16.76 32.31,16.76 33.53,15.54 36.37,15.54 36.47,15.65 39.93,15.65 40.03,15.54 40.74,15.54 40.84,15.65 49.99,15.65 51.31,16.97 52.02,16.97 53.03,17.98 GND.A1 | 15.75,29.77 13.21,29.77 S1.1 | 15.75,29.77 S2.1
  Bottom 0.203: v18.29,30.68 18.29,29.77 18.39,29.67 R21.2 18.49,29.57 21.64,26.42 v21.64,18.9
A2  (via drill 0.41)
  Top 0.203: 45.97,34.59 44.09,36.47 v35.26,36.47 | 45.97,34.59 v46.84,33.73 | v74.47,59.74 73.97,60.25 v65.53,60.25 | v61.67,44.3 v62.89,45.52 | v61.06,34.54 60.96,34.65 58.83,34.65 | 58.83,34.65 46.02,34.65 45.97,34.59 | v74.78,29.46 74.47,29.77 v65.84,29.77 | v63.6,32 61.47,32 58.83,34.65
  Bottom 0.203: v46.84,33.73 46.84,33.33 46.33,32.82 46.33,31.09 IC3.3 | v35.26,36.47 35.05,36.68 35.05,45.82 33.12,47.75 32,47.75 32,45.62 31.9,45.52 IC4.17 | v74.47,59.74 74.37,59.84 74.37,61.06 IC2.17 | v65.53,60.25 62.89,57.61 v62.89,45.52 | v61.67,44.3 61.06,43.69 v61.06,34.54 | v74.78,29.46 76.1,28.14 76.1,27.64 76.81,26.92 U$19.A2 | v63.6,32 v65.84,29.77
D2  (via drill 0.41)
  Top 0.203: v11.99,39.52 14.22,41.76 v22.05,41.76 | v24.49,56.39 29.36,61.27 v53.14,61.27
  Bottom 0.203: v11.99,39.52 11.99,38.41 9.65,38.41 5.99,34.75 R3.2 | v22.05,41.76 22.66,42.37 22.66,54.56 v24.49,56.39 | v53.14,61.27 58.12,66.24 GND.D2
D3  (via drill 0.41)
  Top 0.203: v10.16,43.38 10.46,43.69 19.2,43.69 20.62,45.11 20.62,62.18 39.62,62.18 42.47,65.02 54.36,65.02 55.58,66.24 GND.D3
  Bottom 0.203: v10.16,43.38 5.99,39.22 R4.2
DISP_DATA_OUT  (via drill 0.41)
  Top 0.203: v52.73,48.16 70.21,48.16 70.71,48.67 77.32,48.67 78.54,47.45 SERIAL.6
  Bottom 0.203: v52.73,48.16 50.9,49.99 50.9,60.86 45.52,66.24 GND.D7
GND  (via drill 0.61)
  Top 0.406: 13.31,37.19 10.46,37.19 U$7.K1 | 13.31,37.19 v18.49,37.19 | RESETA.1 13.21,11.48 15.75,11.48 RESET.1 | v13.31,32.21 13.61,31.9 17.07,31.9 v17.37,32.21 | v13.31,37.08 13.31,37.19 | X1.11 109.22,47.85 v102.92,47.85 102.31,47.24 v92.66,47.24 | v111.76,53.44 109.22,53.44 X1.13 109.12,53.44 v106.38,53.44 | v106.38,62.79 v96.83,62.79 | X1.G2 v106.48,60.35 | v68.48,23.88 68.78,23.57 74.47,23.57 75.79,24.89 76.71,24.89 U$19.L3 76.91,24.89 79.05,24.89 U$19.L2 79.25,24.89 v80.97,24.89 81.28,25.2 84.53,25.2 84.63,25.3 91.44,25.3 91.64,25.09 91.64,23.98 92.56,23.98 K4.P2 | v56.29,27.13 67.16,27.13 67.46,26.82 68.48,26.82 v68.58,26.92 | v78.84,55.68 v82.7,55.68 | v43.48,22.96 v48.36,22.96 | v40.44,19.71 v30.99,19.71 v18.59,19.71 | GND.GND@1 42.88,18.09 40.44,18.09 GND.GND@0 | v36.07,16.36 v40.44,16.36 49.28,16.36 v49.58,16.66 | v102.92,23.06 109.22,23.06 X1.2 | v111.76,20.22 111.66,20.32 110.64,20.32 | 110.64,20.32 109.22,20.32 X1.1 | v110.64,20.22 110.64,20.32 | v52.32,8.23 53.65,8.23 53.95,7.92 67.46,7.92 v67.77,8.23 v83.11,8.23 | v83.72,43.18 v80.97,43.18 | v83.21,6.6 v92.46,6.6 92.96,7.11 100.69,7.11 U$15.P$1 | v92.46,44.81 83.72,44.81 SERIAL.1 | v102.92,19.1 102.62,19.41 92.96,19.41 v92.66,19.1 | v92.46,52.73 v82.8,52.73 | v32.31,42.67 32.41,42.57 41.25,42.57 v41.35,42.67 v53.85,42.67 | B10.1 56.08,40.44 57.2,39.32 67.36,39.32 68.48,40.44 B11.1 68.68,40.44 70.71,38.41 91.14,38.41 92.56,36.98 K6.P2 | B15.1 43.48,59.44 42.37,58.32 33.63,58.32 v31.8,56.49 31.7,56.59 31.5,56.59 v28.65,59.44 | v66.34,66.85 v73.05,66.85 73.15,66.95 75.59,66.95 | v77.62,67.67 76.91,66.95 75.59,66.95
  Top 0.406: v75.59,66.85 75.59,66.95
  Bottom 0.305: IC3.25 46.86,25.2 46.86,24.14 47,24 48.36,24
  Bottom 0.406: IC4.10 30.58,52.83 30.58,53.65 30.89,53.95 30.89,54.76 31.09,54.97 C4.1 31.09,55.17 31.8,55.88 v31.8,56.49 | v18.49,37.19 18.49,40.44 B7.1 | 18.49,19.71 v18.49,18.09 18.39,17.98 18.39,15.95 14.22,15.95 11.48,13.21 | 18.49,19.71 18.49,21.34 B1.1 18.49,21.54 18.49,22.86 18.39,22.96 18.39,27.84 R21.1 18.19,27.84 18.19,28.14 17.48,28.85 17.48,32.11 v17.37,32.21 | v13.31,37.08 13.01,36.78 13.01,32.51 v13.31,32.21 | X1.24 X1.25 v111.76,53.44 | X1.13 X1.12 X1.11 | v102.92,47.85 102.92,40.54 B14.1 | v96.83,62.79 97.13,63.09 97.13,66.45 96.52,66.45 C1.1 96.52,66 99,66 99,70 U$18.P$1 | 106.38,60.35 106.38,57.81 POT1.3 106.38,57.61 v106.38,53.44 | 106.38,60.35 v106.38,62.79 | v106.48,60.35 106.38,60.35 | IC3.14 53.44,31.09 55.07,31.09 55.07,30.07 C5.2 55.27,29.97 56.19,29.06 56.19,27.13 | 56.19,27.13 56.19,23.06 55.98,22.86 55.98,21.54 B4.1 | v80.97,24.89 80.97,21.54 B6.1 | B5.1 68.48,21.54 v68.48,23.88 68.58,23.98 v68.58,26.92 | v56.29,27.13 56.19,27.13 | v82.7,55.68 82.7,52.73 | 82.7,52.73 82.7,49.68 C3.2 | v78.84,55.68 77.72,55.68 C7.2 77.52,55.68 77.22,55.68 77.22,58.93 75.59,60.55 75.59,61.06 IC2.15 75.59,61.27 v75.59,66.85 | v48.36,22.96 48.36,24 48.36,24.49 48.26,24.59 48.26,25.2 IC3.23 | v43.48,22.96 43.48,21.54 B3.1 43.48,21.34 43.48,19.91 42.98,19.41 42.98,18.09 GND.GND@1 | OK4.7 35.15,6.6 36.78,6.6 36.78,11.28 36.37,11.68 35.15,11.68 OK4.5 36.07,11.79 v36.07,16.36 | v30.99,19.71 30.99,21.44 B2.1 | v40.44,19.71 40.44,18.09 GND.GND@0 40.44,17.88 v40.44,16.36 | X1.15 X1.14 v111.76,20.22 | v102.92,23.06 102.92,21.54 B13.1 102.92,21.34 v102.92,19.1 | X1.2 X1.1 | v110.64,20.22 110.54,20.12 110.54,13.31 X1.G1
  Bottom 0.406: 52.22,8.23 52.22,11.28 51.82,11.68 50.6,11.68 OK3.5 50.39,11.68 49.68,11.68 49.58,11.79 v49.58,16.66 | 52.22,8.23 52.22,6.6 50.6,6.6 OK3.7 | 67.67,8.23 67.67,11.28 67.26,11.68 66.04,11.68 OK2.5 | 67.67,8.23 67.67,6.6 66.04,6.6 OK2.7 | v52.32,8.23 52.22,8.23 | v67.77,8.23 67.67,8.23 | v80.97,43.18 80.97,40.54 B12.1 | v83.72,43.18 83.72,44.81 SERIAL.1 | 92.56,52.73 92.56,50.09 K7.P2 92.56,49.89 92.56,48.56 K8.P1 92.56,48.36 92.56,47.24 | 92.56,52.73 92.56,54.97 K7.P1 | 83.11,6.6 81.48,6.6 OK1.7 | 83.11,6.6 v83.11,8.23 83.11,11.28 82.7,11.68 81.48,11.68 OK1.5 | 92.56,6.6 92.56,9.35 K1.P1 92.56,9.55 92.56,10.87 K2.P2 92.56,11.07 92.56,15.85 K2.P1 92.56,16.05 92.56,17.37 K3.P2 92.56,17.58 92.56,19.1 | 92.56,6.6 92.56,4.47 K1.P2 | 92.56,19.1 92.56,22.35 K3.P1 92.56,22.55 92.56,23.88 K4.P2 92.56,24.08 92.56,28.85 K4.P1 92.56,29.06 92.56,30.38 K5.P2 92.56,30.58 92.56,35.36 K5.P1 92.56,35.56 92.56,36.88 K6.P2 92.56,37.08 92.56,41.86 K6.P1 92.56,42.06 92.56,43.38 K8.P2 92.56,43.59 92.56,44.81 | v83.21,6.6 83.11,6.6 | v92.46,6.6 92.56,6.6 | 92.56,44.81 92.56,47.24 | v92.46,44.81 92.56,44.81 | v92.66,19.1 92.56,19.1 | v82.8,52.73 82.7,52.73 | v92.46,52.73 92.56,52.73 | v92.66,47.24 92.56,47.24 | v18.59,19.71 18.49,19.71 | 11.48,13.21 7.21,17.48 5.59,17.48 U$20.P$1 | 11.48,13.21 13.21,11.48 RESETA.1 | v32.31,42.67 32.31,41.76 31.09,40.54 B8.1 | v41.35,42.67 43.48,40.54 B9.1 | v53.85,42.67 55.98,40.54 B10.1 | v28.65,59.44 28.65,64.01 26.42,66.24 GND.GND@2 26.42,69 8,69 8,70 U$21.P$1 | 66.14,66.85 66.14,65.73 58.73,58.32 56.08,58.32 56.08,59.44 B16.1 | 66.14,66.85 66.14,67.16 65.23,68.07 C2.1 65.02,68.07 45.31,68.07 44.09,66.85 44.09,65.73 46.74,63.09 46.74,58.32 44.7,58.32 43.59,59.44 B15.1
  Bottom 0.406: v73.05,66.85 73.05,68.28 IC2.10 | v66.34,66.85 66.14,66.85 | v77.62,67.67 77.62,68.38 83.62,68.38 IC1.9
  pour Top: 0,0 119,0 119,74 0,74
  pour Bottom: 0,0 119,0 119,74 0,74
GPA0  (via drill 0.41)
  Top 0.203: v29.16,44.09 27.53,42.47 11.38,42.47 2.13,33.22 2.13,13.41 15.44,13.41 16.46,14.43 B1.2
  Bottom 0.203: v29.16,44.09 29.16,45.31 29.26,45.41 IC4.21
GPA1
  Bottom 0.203: IC4.22 28.55,45.41 28.55,44.5 25.91,41.86 25.91,17.58 28.96,14.53 B2.2
GPA2  (via drill 0.41)
  Top 0.203: v26.01,44.09 24.79,42.88 11.18,42.88 1.73,33.43 1.73,8.94 19.81,8.94 24.69,13.82 26.11,13.82 26.72,13.21 40.23,13.21 41.45,14.43 B3.2
  Bottom 0.203: v26.01,44.09 27.33,44.09 27.94,44.7 27.94,45.41 IC4.23
GPA3  (via drill 0.41)
  Top 0.203: v27.43,46.84 29.06,45.21 v60.66,45.21 | v60.35,21.95 58.62,20.22 v55.37,20.22
  Bottom 0.203: v27.43,46.84 27.43,45.52 IC4.24 | v60.66,45.21 60.35,44.91 v60.35,21.95 | v55.37,20.22 54.36,19.2 54.36,14.83 54.05,14.53 B4.2
GPA4  (via drill 0.41)
  Top 0.203: v27.33,47.75 51.31,47.75 53.24,45.82 60.05,45.82 60.35,46.13 v61.27,46.13 | v62.48,19.61 62.79,19.3 63.8,19.3 v66.24,16.87
  Bottom 0.203: v27.33,47.75 26.72,47.14 26.72,45.52 IC4.25 | v61.27,46.13 62.48,44.91 v62.48,19.61 | v66.24,16.87 66.45,16.66 66.45,14.53 B5.2
GPA5  (via drill 0.41)
  Top 0.203: v26.11,47.75 26.82,48.46 51.41,48.46 53.34,46.53 v53.54,46.53 | v59.23,29.77 60.55,28.45 v74.78,28.45
  Bottom 0.203: v26.11,47.75 26.11,45.52 IC4.26 | v53.54,46.53 59.54,40.54 59.54,30.07 v59.23,29.77 | v74.78,28.45 75.69,27.53 75.69,17.78 78.94,14.53 B6.2
GPA6  (via drill 0.41)
  Top 0.203: v25.09,38 24.99,37.9 v20.93,37.9
  Bottom 0.203: v25.09,38 25.3,38.2 25.3,45.41 IC4.27 | v20.93,37.9 16.56,33.53 B7.2
GPA7  (via drill 0.41)
  Top 0.203: v25.2,33.73 26.52,32.41 27.94,32.41 28.96,33.43 B8.2
  Bottom 0.203: v25.2,33.73 25.2,35.36 24.38,36.17 24.38,45.11 24.69,45.41 IC4.28
GPB0  (via drill 0.61)
  Top 0.406: v23.88,35.56 24.69,34.75 40.23,34.75 41.45,33.53 B9.2
  Bottom 0.406: v23.88,35.56 23.88,51.92 24.69,52.73 IC4.1
GPB1  (via drill 0.41)
  Top 0.203: v48.77,38.71 v23.06,38.71
  Bottom 0.203: v23.06,38.71 23.06,53.85 25.09,53.85 25.3,53.65 25.3,52.83 IC4.2 | v48.77,38.71 53.95,33.53 B10.2
GPB2  (via drill 0.41)
  Top 0.203: v25.2,47.55 27.94,44.81 44.09,44.81 v45.21,43.69 | v53.54,35.36 53.65,35.26 64.72,35.26 66.45,33.53 B11.2
  Bottom 0.203: v25.2,47.55 25.2,48.46 25.91,49.17 25.91,52.63 26.01,52.73 IC4.3 | v53.54,35.36 v45.21,43.69
GPB3  (via drill 0.41)
  Top 0.203: v30.18,46.84 30.89,46.13 v44.6,46.13 | v49.68,40.23 52.73,37.19 75.29,37.19 78.94,33.53 B12.2
  Bottom 0.203: v30.18,46.84 26.82,50.19 26.82,52.63 26.72,52.73 IC4.4 | v44.6,46.13 49.68,41.05 v49.68,40.23
GPB4  (via drill 0.41)
  Top 0.203: v27.43,54.15 28.55,55.27 46.13,55.27 47.04,56.19 72.85,56.19 73.15,55.88 77.52,55.88 79.45,53.95 v81.89,53.95 | v85.45,14.83 86.87,13.41 99.77,13.41 100.79,14.43 B13.2
  Bottom 0.203: v27.43,54.15 27.43,52.83 IC4.5 | v81.89,53.95 81.89,48.46 82.4,47.95 82.4,42.67 84.73,40.34 84.73,26.62 85.65,25.7 85.65,15.04 v85.45,14.83
GPB5  (via drill 0.41)
  Top 0.203: v28.55,51.41 29.06,51.92 38.51,51.92 39.12,51.31 v48.06,51.31 | v50.6,40.34 53.03,37.9 87.58,37.9 89.51,35.97 89.51,34.65 99.67,34.65 100.79,33.53 B14.2
  Bottom 0.203: v28.55,51.41 28.04,51.92 28.04,52.73 IC4.6 | v48.06,51.31 50.6,48.77 v50.6,40.34
GPB6  (via drill 0.41)
  Top 0.203: v28.45,54.15 28.96,53.65 40.34,53.65 41.45,52.53 B15.2
  Bottom 0.203: v28.45,54.15 28.55,54.05 28.55,52.83 IC4.7
GPB7  (via drill 0.41)
  Top 0.203: v30.38,49.99 30.48,49.89 v52.02,49.89
  Bottom 0.203: v30.38,49.99 29.36,51 29.36,52.73 IC4.8 | v52.02,49.89 53.95,51.82 53.95,52.43 B16.2
I2C_SCL  (via drill 0.41)
  Top 0.203: v46.33,26.31 44.5,28.14 v36.27,28.14 | v77.62,62.38 71.73,62.38 v70.92,63.2 69.7,63.2 67.46,65.43 66.04,65.43 63.91,67.56 20.02,67.56 18.8,66.34 JP4.2 | v31.39,51.21 30.89,50.7 26.31,50.7 v22.05,54.97
  Bottom 0.203: v46.33,26.31 46.33,25.3 IC3.26 | v36.27,28.14 35.66,28.75 35.66,30.99 35.97,31.29 35.97,47.85 31.95,51.87 | 31.95,51.87 31.9,51.92 31.9,52.73 IC4.12 | JP4.2 18.8,64.62 20.32,63.09 R2.1 20.42,62.99 21.23,62.18 21.23,61.27 22.05,60.45 v22.05,54.97 | v70.92,63.2 74.27,66.55 74.27,68.28 IC2.12 | v77.62,62.38 81.08,62.38 81.08,47.45 SERIAL.4 | 31.95,51.87 31.39,51.31 v31.39,51.21
I2C_SDA  (via drill 0.41)
  Top 0.203: v74.78,63.8 82.4,63.8 83.52,62.69 83.52,53.54 82.5,53.54 79.86,50.9 79.86,49.07 | 79.86,49.07 79.86,44.91 81.08,44.91 SERIAL.3 | v45.62,28.04 44.6,29.06 v36.37,29.06 | v30.38,62.89 29.46,63.8 23.77,63.8 21.34,66.24 JP4.1 | 79.86,49.07 67.46,49.07 66.95,48.56 54.36,48.56 52.32,50.6 v36.37,50.6
  Bottom 0.203: v74.78,63.8 74.78,67.16 74.88,67.26 74.88,68.28 IC2.13 | JP4.1 21.34,64.52 22.76,63.09 R1.1 | v45.62,28.04 45.62,25.3 IC3.27 | v36.37,29.06 v36.37,50.6 36.37,51 33.53,53.85 32.61,53.85 | 32.61,53.85 32.61,52.83 IC4.13 | v30.38,62.89 32.61,60.66 32.61,53.85
L0
  Bottom 0.203: R37.1 20.42,16.46 20.42,14.53 B1.L1 20.32,14.53 18.59,14.53 B1.L2
L1
  Top 0.203: B2.L2 31.09,14.53 32.92,14.53 B2.L1
  Bottom 0.203: R36.1 33.02,16.05 33.02,14.53 B2.L1
L2
  Top 0.203: B3.L2 43.59,14.53 45.41,14.53 B3.L1
  Bottom 0.203: R35.1 45.62,16.05 45.52,15.95 45.52,14.53 B3.L1
L3
  Top 0.203: B4.L2 56.08,14.53 57.91,14.53 B4.L1
  Bottom 0.203: R34.1 58.01,16.05 58.01,14.53 B4.L1
L4
  Top 0.203: B5.L2 68.58,14.53 70.41,14.53 B5.L1
  Bottom 0.203: R33.1 70.51,16.05 70.51,14.53 B5.L1
L5
  Top 0.203: B6.L2 81.08,14.53 82.91,14.53 B6.L1
  Bottom 0.203: R32.1 83.01,16.15 83.01,14.53 B6.L1
L6
  Top 0.203: B7.L2 18.59,33.53 20.42,33.53 B7.L1
  Bottom 0.203: R31.1 20.52,31.8 20.52,33.43 B7.L1
L7
  Top 0.203: B8.L2 31.09,33.53 32.92,33.53 B8.L1
  Bottom 0.203: R30.1 33.12,31.8 33.02,31.9 33.02,33.43 B8.L1
L8
  Top 0.203: B9.L2 43.59,33.53 45.41,33.53 B9.L1
  Bottom 0.203: R29.1 45.62,35.05 45.52,34.95 45.52,33.53 B9.L1
L9
  Top 0.203: B10.L2 56.08,33.53 57.91,33.53 B10.L1
  Bottom 0.203: R28.1 58.01,31.9 58.01,33.43 B10.L1
L10
  Top 0.203: B11.L2 68.58,33.53 70.41,33.53 B11.L1
  Bottom 0.203: R27.1 70.51,31.8 70.51,33.43 B11.L1
L11
  Top 0.203: B12.L2 81.08,33.53 82.91,33.53 B12.L1
  Bottom 0.203: R26.1 83.01,33.43 B12.L1
L12
  Top 0.203: B13.L2 102.92,14.53 104.85,14.53 B13.L1
  Bottom 0.203: R25.1 106.48,16.76 104.95,15.24 104.95,14.53 B13.L1
L13
  Top 0.203: B14.L2 102.92,33.53 104.85,33.53 B14.L1
  Bottom 0.203: R24.1 105.66,29.87 104.95,30.58 104.95,33.43 B14.L1
L14
  Top 0.203: B15.L2 43.59,52.53 45.41,52.53 B15.L1
  Bottom 0.203: R23.1 45.52,50.8 45.52,52.43 B15.L1
L15
  Top 0.203: B16.L2 56.08,52.53 57.91,52.53 B16.L1
  Bottom 0.203: R22.1 58.01,50.9 58.01,52.43 B16.L1
N$1
  Bottom 0.305: K1.S1 94.79,9.45 94.18,8.84 94.18,8.13 94.59,7.72 97.33,7.72 97.33,8.43 99.47,10.57 109.12,10.57 109.32,10.36 113.49,10.36 113.49,44.7 111.76,46.43 X1.23
N$2  (via drill 0.41)
  Top 0.203: v52.63,32.11 52.32,32.41 35.76,32.41 v35.26,32.92
  Bottom 0.203: v52.63,32.11 52.63,31.19 52.73,31.09 IC3.13 | v35.26,32.92 35.05,32.72 35.05,31.9 34.95,31.8 R30.2
N$4  (via drill 0.41)
  Top 0.203: v95.71,56.29 102.72,49.28 110.13,49.28 111.86,47.55 113.08,47.55 115.32,45.31 115.32,3.35 88.29,3.35 87.27,4.37 K1.16
  Bottom 0.203: v95.71,56.29 93.78,58.22 IC1.18
N$5  (via drill 0.41)
  Top 0.203: v66.34,68.68 66.55,68.48 83.92,68.48 v85.45,66.95
  Bottom 0.203: v66.34,68.68 66.34,68.38 67.16,68.38 IC2.1 | v85.45,66.95 86.06,66.34 86.06,60.15 84.23,58.32 83.72,58.32 IC1.1
N$6
  Top 0.305: K2.S1 94.89,16.05 97.13,18.29 105.56,18.29 109.12,21.84 110.34,21.84 111.76,23.27 112.27,23.27 114.4,25.4 114.4,43.69 111.76,43.69 X1.22
N$7
  Bottom 0.203: R4.1 7.62,39.22 10.36,39.22 10.36,39.62 U$7.A2
N$9  (via drill 0.41)
  Top 0.203: v87.38,53.54 v92.15,58.32 | v88.8,32.72 v85.65,35.87
  Bottom 0.203: v92.15,58.32 92.15,59.54 93.67,59.54 IC1.17 | v87.38,53.54 85.65,51.82 v85.65,35.87 | v88.8,32.72 88.49,32.41 88.49,19.71 88.09,19.3 88.09,11.79 87.27,10.97 K2.16
N$10
  Top 0.305: K3.S1 94.89,22.55 96.93,24.59 110.34,24.59 111.76,26.01 112.27,26.01 113.89,27.64 113.89,40.95 111.76,40.95 X1.21
N$11
  Bottom 0.203: R3.1 7.62,34.65 10.36,34.65 U$7.A3
N$13  (via drill 0.41)
  Top 0.203: v95.3,57.71 93.47,55.88 93.47,50.9 v91.75,50.9 | v89.1,19.3 87.27,17.48 K3.16
  Bottom 0.203: v95.3,57.71 95.3,60.76 93.78,60.76 IC1.16 | v91.75,50.9 91.34,50.49 91.34,21.54 v89.1,19.3
N$14
  Top 0.305: X1.20 112.88,38.2 112.88,34.95 112.27,34.34 111.76,34.34 110.34,32.92 109.22,32.92 105.66,29.36 95.2,29.36 94.89,29.06 K4.S1
N$17  (via drill 0.41)
  Top 0.203: v93.47,41.25 92.05,39.83 v88.8,39.83
  Bottom 0.203: v93.47,41.25 93.47,43.38 96.42,46.33 96.42,62.08 93.78,62.08 IC1.15 | v88.8,39.83 88.09,39.12 88.09,24.79 87.27,23.98 K4.16
N$18
  Top 0.305: X1.19 94.89,35.46 K5.S1
N$19  (via drill 0.41)
  Top 0.203: v49.17,36.98 48.97,37.19 v23.06,37.19
  Bottom 0.203: v49.17,36.98 49.17,34.54 52.02,31.7 52.02,31.19 52.12,31.09 IC3.12 | v23.06,37.19 22.55,36.68 22.55,32.11 22.25,31.8 R31.2
N$21  (via drill 0.41)
  Top 0.203: v95.4,63.3 93.07,60.96 v90.63,60.96 | v89.2,30.89 88.8,30.48 87.27,30.48 K5.16
  Bottom 0.203: v95.4,63.3 93.78,63.3 IC1.14 | v90.63,60.96 89.51,59.84 89.51,31.19 v89.2,30.89
N$22  (via drill 0.3)
  Top 0.305: v112.06,36.78 111.56,36.78 110.34,38 109.22,38 105.56,41.66 95.2,41.66 94.89,41.96 K6.S1
  Bottom 0.305: v112.06,36.78 112.88,35.97 112.88,33.83 111.76,32.72 X1.18
N$23  (via drill 0.41)
  Top 0.203: v50.39,28.25 49.58,29.06 49.58,30.89 71.93,30.89 72.24,31.19 79.45,31.19 v80.87,29.77
  Bottom 0.203: v50.39,28.25 51.71,29.57 51.71,30.28 51.61,30.38 51.61,30.89 51.51,30.99 IC3.11 | v80.87,29.77 84.63,26.01 84.63,16.26 R32.2
N$25  (via drill 0.41)
  Top 0.203: v88.8,56.9 v92.15,60.25
  Bottom 0.203: v92.15,60.25 92.15,64.62 93.67,64.62 IC1.13 | v88.8,56.9 88.49,56.59 88.49,40.54 87.27,39.32 87.27,36.98 K6.16
N$26  (via drill 0.3)
  Top 0.305: v104.04,48.67 101.19,48.67 94.89,54.97 K7.S1
  Bottom 0.305: v104.04,48.67 109.22,43.48 110.64,43.48 110.64,31.09 111.76,29.97 X1.17
N$29  (via drill 0.41)
  Top 0.203: v91.34,51.92 90.32,50.9 88.19,50.9 87.27,49.99 K7.16
  Bottom 0.203: v91.34,51.92 91.34,65.84 93.67,65.84 IC1.12
N$30  (via drill 0.3)
  Top 0.305: v97.03,47.95 95.4,47.95 94.89,48.46 K8.S1 | v100.48,27.23 111.76,27.23 X1.16
  Bottom 0.305: v97.03,47.95 97.43,47.55 97.43,30.28 v100.48,27.23
N$31  (via drill 0.41)
  Top 0.203: v51,29.97 51.51,30.48 v72.54,30.48
  Bottom 0.203: v51,29.97 51,30.89 50.9,30.99 IC3.10 | v72.54,30.48 72.34,30.28 72.34,16.15 R33.2
N$33
  Bottom 0.203: IC1.11 93.67,67.16 88.09,67.16 88.09,44.3 87.27,43.48 K8.16
N$34  (via drill 0.41)
  Top 0.203: v67.87,64.01 71.22,60.66 75.89,60.66 78.03,58.52 v82.09,58.52
  Bottom 0.203: v67.87,64.01 67.87,68.28 IC2.2 | v82.09,58.52 83.11,59.54 83.62,59.54 IC1.2
N$35  (via drill 0.41)
  Top 0.203: v66.65,69.6 67.36,68.89 84.63,68.89 86.16,67.36 86.16,61.98 v85.34,61.98
  Bottom 0.203: v66.65,69.6 67.97,69.6 68.38,69.19 68.38,68.38 IC2.3 | v85.34,61.98 84.23,60.86 83.72,60.86 IC1.3
N$36  (via drill 0.41)
  Top 0.203: v68.99,66.04 66.04,66.04 65.53,66.55 65.53,67.77 v76.4,67.77
  Bottom 0.203: v68.99,66.04 68.99,68.17 69.09,68.28 IC2.4 | v76.4,67.77 81.99,62.18 83.62,62.18 IC1.4
N$37  (via drill 0.41)
  Top 0.203: v69.9,65.23 72.03,63.09 v82.09,63.09
  Bottom 0.203: v69.9,65.23 69.9,68.17 69.8,68.28 IC2.5 | v82.09,63.09 83.62,63.09 83.62,63.3 IC1.5
N$38  (via drill 0.41)
  Top 0.203: v71.42,64.72 71.63,64.52 v82.09,64.52
  Bottom 0.203: v71.42,64.72 70.41,65.73 70.41,68.28 IC2.6 | v82.09,64.52 83.62,64.52 83.62,64.62 IC1.6
N$39  (via drill 0.41)
  Top 0.203: v71.12,66.04 71.83,65.33 v81.58,65.33
  Bottom 0.203: v71.12,66.04 71.12,68.28 IC2.7 | v81.58,65.33 83.62,65.33 83.62,65.84 IC1.7
N$40  (via drill 0.41)
  Top 0.203: v85.34,66.04 v72.34,66.04
  Bottom 0.203: v72.34,66.04 71.83,66.55 71.83,68.17 71.73,68.28 IC2.8 | v85.34,66.04 84.23,67.16 83.72,67.16 IC1.8
N$47
  Bottom 0.203: R13.2 69.8,9.04 71.83,9.04 71.83,9.14 OK1.3
N$48
  Bottom 0.203: R14.2 69.9,4.17 71.83,4.17 OK1.1
N$49  (via drill 0.3)
  Top 0.152: v79.45,6.6 80.67,5.38 97.84,5.38 99.47,3.76 104.95,3.76 114.91,13.72 114.91,45.11 X1.10
  Bottom 0.152: v79.45,6.6 71.93,6.6 OK1.2
N$50
  Bottom 0.203: R15.2 54.56,4.17 56.39,4.17 OK2.1
N$51
  Bottom 0.203: IC2.21 71.73,61.06 71.83,60.96 71.83,51.31 74.07,49.07 74.07,12.9 80.06,6.91 80.06,5.49 81.38,4.17 OK1.8
N$52
  Bottom 0.203: R16.2 54.56,9.04 56.39,9.04 56.39,9.14 OK2.3
N$53
  Bottom 0.203: R17.2 39.12,4.17 40.95,4.17 OK3.1
N$54
  Bottom 0.203: R18.2 39.12,9.25 40.95,9.25 OK3.3
N$55  (via drill 0.3)
  Top 0.152: v47.65,6.71 49.99,9.04 86.46,9.04 86.87,8.64 92.96,8.64 v93.67,9.35 | v96.72,32.61 96.93,32.41 107.59,32.41 109.22,34.04 X1.6
  Bottom 0.152: v47.65,6.71 41.05,6.71 OK3.2 | v93.67,9.35 93.88,9.55 93.88,26.92 96.72,29.77 v96.72,32.61
N$56
  Bottom 0.203: R19.2 23.47,4.17 25.6,4.17 OK4.1
N$57
  Bottom 0.203: R20.2 23.57,9.25 25.6,9.25 OK4.3
N$58  (via drill 0.41)
  Top 0.203: v50.29,29.36 51.1,28.55 v59.23,28.55
  Bottom 0.203: v50.29,29.36 50.29,30.89 50.19,30.99 IC3.9 | v59.23,28.55 59.23,18.8 59.44,18.59 59.44,16.46 59.74,16.15 R34.2
N$59  (via drill 0.41)
  Top 0.203: v46.23,23.77 v49.38,26.92
  Bottom 0.203: v49.38,26.92 49.38,30.89 49.48,30.99 IC3.8 | v46.23,23.77 47.24,22.76 47.24,16.15 R35.2
N$60  (via drill 0.3)
  Top 0.152: v73.46,26.72 74.47,27.74 100.08,27.74 101.19,28.85 108,28.85 109.42,30.28 110.64,30.28 111.96,31.6 112.17,31.6 113.39,32.82 113.39,39.93 111.25,39.93 109.22,41.96 X1.9
  Bottom 0.152: v73.46,26.72 73.46,13.31 71.93,11.79 OK1.4
N$61  (via drill 0.3)
  Top 0.152: v62.48,6.71 63.2,7.42 92.56,7.42 93.57,8.43 v94.89,8.43
  Bottom 0.152: v62.48,6.71 56.49,6.71 OK2.2 | v94.89,8.43 97.84,11.38 97.84,21.95 104.85,28.96 106.88,28.96 106.88,37.19 109.22,39.52 X1.8
N$62  (via drill 0.3)
  Top 0.152: v61.37,13.61 63.3,15.54 86.46,15.54 86.87,15.14 98.04,15.14 100.69,17.78 v106.58,17.78
  Bottom 0.152: v61.37,13.61 61.37,11.79 56.49,11.79 OK2.4 | v106.58,17.78 107.19,18.39 107.19,28.75 108.1,29.67 108.1,35.66 109.22,36.78 X1.7
N$63  (via drill 0.41)
  Top 0.203: v66.34,58.62 65.02,57.3 v50.19,57.3 | v34.34,44.09 v41.55,44.09 | v34.34,32.92 34.34,30.48 v38.91,30.48 | v36.88,14.94 35.87,13.92 v35.05,13.92
  Bottom 0.203: v66.34,58.62 66.85,59.13 66.85,60.76 67.16,61.06 IC2.28 | v50.19,57.3 47.04,54.15 47.04,49.58 v41.55,44.09 | v34.34,32.92 v34.34,44.09 | v38.91,30.48 38.61,30.18 38.61,23.27 36.58,21.23 36.58,16.97 36.88,16.66 v36.88,14.94 | v35.05,13.92 33.83,12.7 33.83,10.46 35.05,9.25 OK4.6
N$64  (via drill 0.3)
  Top 0.152: v42.47,13.21 42.67,13.01 103.94,13.01 v104.24,13.31
  Bottom 0.152: v42.47,13.21 41.05,11.79 OK3.4 | v104.24,13.31 107.59,13.31 107.59,28.45 109.22,30.07 X1.5
N$65  (via drill 0.3)
  Top 0.152: v28.75,10.26 30.68,12.19 104.95,12.19 v112.78,20.02
  Bottom 0.152: v28.75,10.26 28.75,9.75 25.7,6.71 OK4.2 | v112.78,20.02 112.88,20.12 112.88,27.53 111.56,28.85 109.22,28.85 X1.4
N$66  (via drill 0.3)
  Top 0.152: v27.23,11.79 28.04,12.6 104.44,12.6 v108.31,16.46
  Bottom 0.152: v27.23,11.79 25.7,11.79 OK4.4 | v108.31,16.46 108.1,16.66 108.1,24.59 109.22,25.7 X1.3
N$67
  Bottom 0.203: IC3.7 48.87,31.09 48.77,31.19 48.77,36.37 48.16,36.98 38.2,36.98 38.2,24.89 35.66,22.35 35.66,20.22 34.04,18.59 34.04,16.87 34.75,16.15 R36.2
N$68  (via drill 0.41)
  Top 0.203: v73.25,27.74 72.34,26.82 v71.12,26.82 | v71.12,25.4 71.53,24.99 v74.78,24.99
  Bottom 0.203: v73.25,27.74 73.25,49.28 71.12,51.41 71.12,61.06 IC2.22 | v71.12,25.4 v71.12,26.82 | v74.78,24.99 75.29,24.49 75.29,14.63 80.67,9.25 81.38,9.25 OK1.6
N$69  (via drill 0.41)
  Top 0.203: v70.31,46.63 67.06,43.38 v61.77,43.38
  Bottom 0.203: v70.31,46.63 70.31,60.96 70.41,61.06 IC2.23 | v61.77,43.38 61.77,33.73 61.06,33.02 61.06,19.51 61.98,18.59 61.98,8.13 65.94,4.17 OK2.8
N$70  (via drill 0.41)
  Top 0.203: v71.73,49.78 v68.99,52.53 | v72.54,34.04 70.51,32 v67.56,32
  Bottom 0.203: v68.99,52.53 68.99,57.3 69.39,57.71 69.39,59.84 69.7,60.15 69.7,61.06 IC2.24 | v71.73,49.78 72.54,48.97 v72.54,34.04 | v67.56,32 66.55,30.99 66.55,25.09 63.4,21.95 63.4,21.03 64.52,19.91 64.52,16.05 63.4,14.94 63.4,11.79 65.94,9.25 OK2.6
N$71  (via drill 0.41)
  Top 0.203: v65.23,55.47 v67.46,55.47 | v61.77,32.72 v63.6,34.54 | v61.77,20.22 61.77,18.8 61.98,18.59 61.98,16.56 51.51,16.56 48.87,13.92 v48.77,13.92
  Bottom 0.203: v67.46,55.47 68.38,56.39 68.38,59.33 68.99,59.94 68.99,60.96 69.09,61.06 IC2.25 | v65.23,55.47 63.6,53.85 63.6,44.7 63.91,44.4 63.91,41.45 63.4,40.95 63.4,34.75 v63.6,34.54 | v61.77,20.22 v61.77,32.72 | v48.77,13.92 48.26,13.41 48.26,6.4 50.49,4.17 OK3.8
N$72  (via drill 0.41)
  Top 0.203: v67.67,57.61 66.65,56.59 43.99,56.59 43.08,55.68 v21.34,55.68 | v21.84,27.23 v21.84,32.92 | v24.99,13.11 28.45,9.65 v48.97,9.65
  Bottom 0.203: v67.67,57.61 67.67,59.33 68.38,60.05 68.38,61.06 IC2.26 | v21.34,55.68 21.34,41.25 21.84,40.74 v21.84,32.92 | v21.84,27.23 24.99,24.08 v24.99,13.11 | v48.97,9.65 50.49,9.65 50.49,9.25 OK3.6
N$73  (via drill 0.41)
  Top 0.203: v46.63,54.76 v66.85,54.76 | v38.51,39.62 38.3,39.42 21.44,39.42 20.22,38.2 20.22,34.65 v23.27,34.65
  Bottom 0.203: v66.85,54.76 66.75,54.86 66.75,57.71 67.26,58.22 67.26,59.54 67.77,60.05 67.77,61.06 IC2.27 | v46.63,54.76 46.63,50.19 38.41,41.96 38.41,39.73 v38.51,39.62 | v23.27,34.65 25.5,32.41 25.5,14.43 33.83,6.1 33.83,5.38 35.05,4.17 OK4.8
N$74  (via drill 0.41)
  Top 0.203: v48.16,29.97 47.95,29.77 35.76,29.77 29.26,23.27 v24.28,23.27
  Bottom 0.203: v48.16,29.97 48.16,30.99 IC3.6 | v24.28,23.27 22.35,21.34 22.35,16.66 22.25,16.56 R37.2
N$75  (via drill 0.41)
  Top 0.203: v54.25,25.3 54.36,25.4 v57,25.4 | v47.85,36.27 v56.79,36.27
  Bottom 0.203: v54.25,25.3 53.44,25.3 IC3.15 | v57,25.4 58.52,26.92 58.52,30.79 59.13,31.39 59.13,33.93 v56.79,36.27 | v47.85,36.27 47.35,35.76 47.35,35.15 R29.2
N$76  (via drill 0.41)
  Top 0.203: v52.93,29.26 53.44,29.77 v56.59,29.77
  Bottom 0.203: v52.93,29.26 52.93,25.4 52.83,25.3 IC3.16 | v56.59,29.77 56.39,29.97 56.39,31.8 R28.2
N$77  (via drill 0.41)
  Top 0.203: v52.22,26.82 53.34,27.94 58.83,27.94 59.03,27.74 v67.67,27.74
  Bottom 0.203: v52.22,26.82 52.22,25.3 IC3.17 | v67.67,27.74 68.68,28.75 68.68,31.7 R27.2
N$78  (via drill 0.41)
  Top 0.203: v55.37,23.57 55.88,23.06 v78.54,23.06
  Bottom 0.203: v55.37,23.57 52.63,23.57 51.61,24.59 51.61,25.09 51.51,25.2 IC3.18 | v78.54,23.06 80.16,24.69 80.16,30.58 81.28,31.7 R26.2
N$79  (via drill 0.41)
  Top 0.203: v51,22.66 74.27,22.66 76.5,20.42 90.63,20.42 91.85,21.64 96.93,21.64 99.16,23.88 v104.04,23.88
  Bottom 0.203: v51,22.66 51,25.09 50.9,25.2 IC3.19 | v104.04,23.88 105.97,21.95 105.97,17.88 104.95,16.87 R25.2
N$80  (via drill 0.41)
  Top 0.203: v50.29,26.82 51,26.11 76.4,26.11 76.5,26.01 v100.28,26.01
  Bottom 0.203: v50.29,26.82 50.29,25.4 50.19,25.3 IC3.20 | v100.28,26.01 104.04,29.77 R24.2
N$81  (via drill 0.41)
  Top 0.203: v49.89,22.05 48.26,20.42 40.84,20.42 40.74,20.52 40.03,20.52 39.93,20.42 35.26,20.42 v34.95,20.73
  Bottom 0.203: v49.89,22.05 49.68,22.25 49.68,25.09 49.58,25.2 IC3.21 | v34.95,20.73 35.26,21.03 35.26,23.16 37.8,25.7 37.8,44.81 43.69,50.7 R23.2
N$82  (via drill 0.41)
  Top 0.203: v49.17,20.02 49.68,19.51 v59.94,19.51
  Bottom 0.203: v49.17,20.02 49.17,23.27 49.07,23.37 49.07,25.09 48.97,25.2 IC3.22 | v59.94,19.51 59.64,19.81 59.64,27.94 59.94,28.25 59.94,47.24 56.39,50.8 R22.2
RES  (via drill 0.41)
  Top 0.203: RESETA.3 13.21,6.4 15.75,6.4 RESET.3 | v30.58,15.85 30.38,15.65 24.99,15.65 v19,9.65
  Bottom 0.203: v30.58,15.85 32.72,17.98 GND.RES | v19,9.65 15.75,6.4 RESET.3
SDI_MOSI  (via drill 0.41)
  Top 0.203: v74.78,34.14 76.91,32 100.08,32 101.3,30.79 JP2.2
  Bottom 0.203: v74.78,34.14 74.78,46.13 76,47.35 SERIAL.8
SDI_SCLK  (via drill 0.41)
  Top 0.203: v75.89,32 76.3,31.6 97.94,31.6 98.75,30.79 JP2.1
  Bottom 0.203: v75.89,32 75.89,44.7 76,44.81 SERIAL.7
SLIDER_IN  (via drill 0.41)
  Top 0.203: v52.73,15.85 53.03,16.15 63.09,16.15 63.7,16.76 65.13,16.76 v65.23,16.87 | v71.83,40.23 75.08,43.48 77.22,43.48 78.54,44.81 SERIAL.5
  Bottom 0.203: C7.1 75.79,55.68 73.66,55.68 73.66,54.36 POT1.2A 73.66,54.25 75.79,52.12 75.79,49.48 77.32,47.95 77.32,46.13 78.54,44.91 SERIAL.5 | v52.73,15.85 50.6,17.98 GND.A0 | v65.23,16.87 68.78,20.42 71.83,20.42 v71.83,40.23

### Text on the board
_tsilk: SCL SDA
_bsilk: SKAARHOJ 2013 | PCB-CMB-5-SHLD v08-13 | I2C PullUps

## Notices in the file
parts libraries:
SparkFun: Licensing: CC v3.0 Share-Alike You are welcome to use this library for commercial purposes.
